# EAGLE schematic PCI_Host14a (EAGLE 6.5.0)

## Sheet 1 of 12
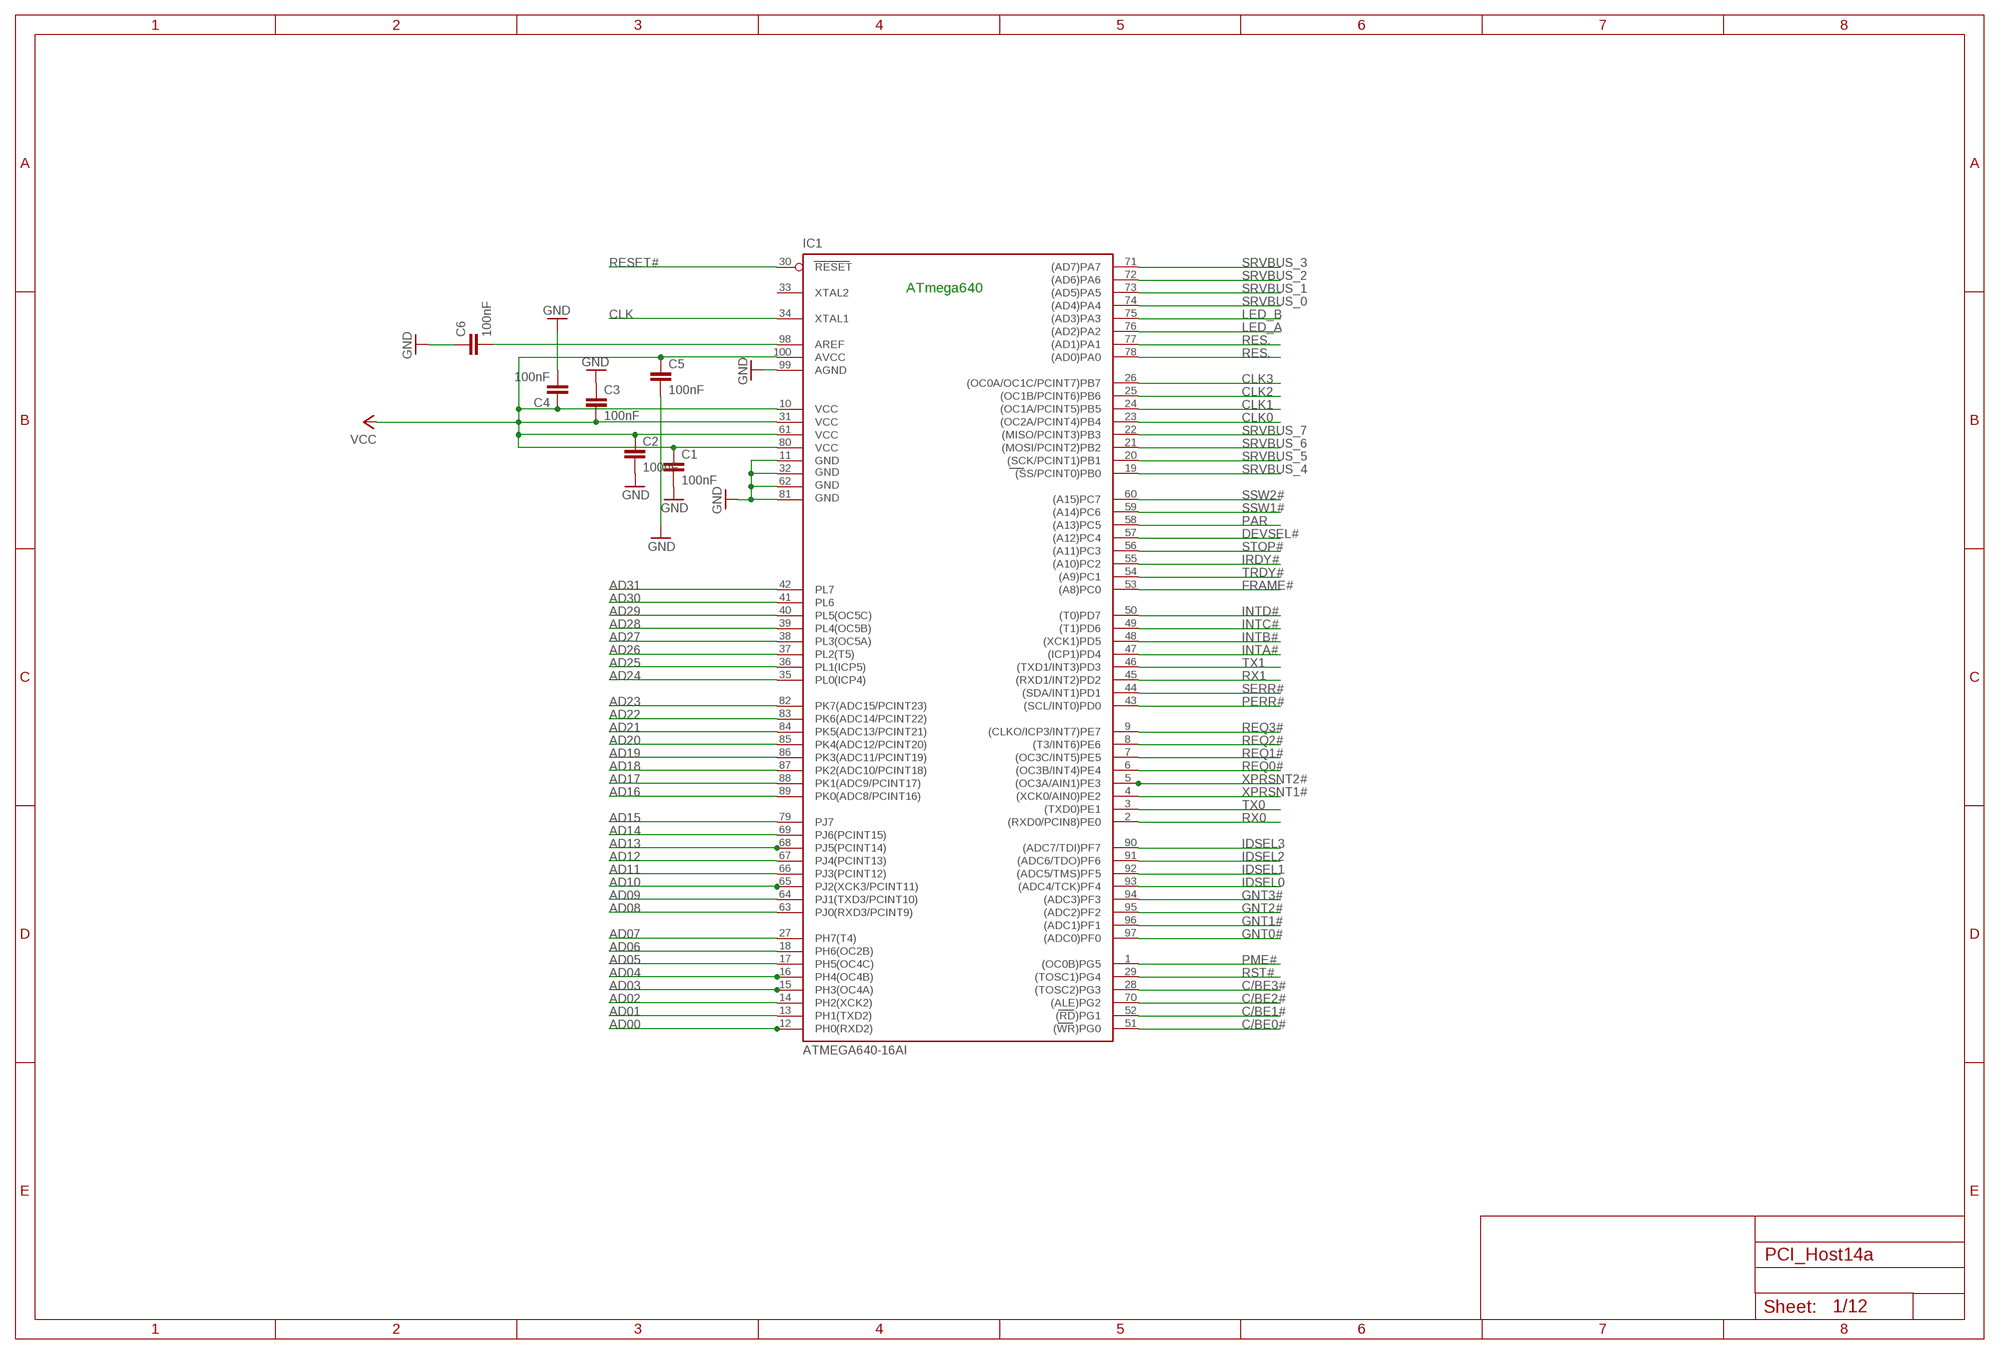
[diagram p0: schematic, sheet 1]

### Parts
C1  100nF  C-EU025-025X050  [C025-025X050]
C2  100nF  C-EU025-025X050  [C025-025X050]
C3  100nF  C-EU025-025X050  [C025-025X050]
C4  100nF  C-EU025-025X050  [C025-025X050]
C5  100nF  C-EU025-025X050  [C025-025X050]
C6  100nF  C-EU025-025X050  [C025-025X050]
IC1  ATMEGA640-16AI  [TQFP100]

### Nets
AD00: IC1.12(PH0(RXD2)) ; also sheet 8
AD01: IC1.13(PH1(TXD2)) ; also sheet 8
AD02: IC1.14(PH2(XCK2)) ; also sheet 8
AD03: IC1.15(PH3(OC4A)) ; also sheet 8
AD04: IC1.16(PH4(OC4B)) ; also sheet 8
AD05: IC1.17(PH5(OC4C)) ; also sheet 8
AD06: IC1.18(PH6(OC2B)) ; also sheet 8
AD07: IC1.27(PH7(T4)) ; also sheet 8
AD08: IC1.63(PJ0(RXD3/PCINT9)) ; also sheet 8
AD09: IC1.64(PJ1(TXD3/PCINT10)) ; also sheet 8
AD10: IC1.65(PJ2(XCK3/PCINT11)) ; also sheet 8
AD11: IC1.66(PJ3(PCINT12)) ; also sheet 8
AD12: IC1.67(PJ4(PCINT13)) ; also sheet 8
AD13: IC1.68(PJ5(PCINT14)) ; also sheet 8
AD14: IC1.69(PJ6(PCINT15)) ; also sheet 8
AD15: IC1.79(PJ7) ; also sheet 8
AD16: IC1.89(PK0(ADC8/PCINT16)) ; also sheet 8
AD17: IC1.88(PK1(ADC9/PCINT17)) ; also sheet 8
AD18: IC1.87(PK2(ADC10/PCINT18)) ; also sheet 8
AD19: IC1.86(PK3(ADC11/PCINT19)) ; also sheet 8
AD20: IC1.85(PK4(ADC12/PCINT20)) ; also sheet 8
AD21: IC1.84(PK5(ADC13/PCINT21)) ; also sheet 8
AD22: IC1.83(PK6(ADC14/PCINT22)) ; also sheet 8
AD23: IC1.82(PK7(ADC15/PCINT23)) ; also sheet 8
AD24: IC1.35(PL0(ICP4)) ; also sheet 8
AD25: IC1.36(PL1(ICP5)) ; also sheet 8
AD26: IC1.37(PL2(T5)) ; also sheet 8
AD27: IC1.38(PL3(OC5A)) ; also sheet 8
AD28: IC1.39(PL4(OC5B)) ; also sheet 8
AD29: IC1.40(PL5(OC5C)) ; also sheet 8
AD30: IC1.41(PL6) ; also sheet 8
AD31: IC1.42(PL7) ; also sheet 8
AREF: C6.2 IC1.98(AREF)
C/BE0#: IC1.51((WR)PG0) ; also sheet 8
C/BE1#: IC1.52((RD)PG1) ; also sheet 8
C/BE2#: IC1.70((ALE)PG2) ; also sheet 8
C/BE3#: IC1.28((TOSC2)PG3) ; also sheet 8
CLK: IC1.34(XTAL1) ; also sheet 3
CLK0: IC1.23((OC2A/PCINT4)PB4) ; also sheet 8
CLK1: IC1.24((OC1A/PCINT5)PB5) ; also sheet 8
CLK2: IC1.25((OC1B/PCINT6)PB6) ; also sheet 8
CLK3: IC1.26((OC0A/OC1C/PCINT7)PB7) ; also sheet 8
DEVSEL#: IC1.57((A12)PC4) ; also sheet 2,8
FRAME#: IC1.53((A8)PC0) ; also sheet 2,8
GND: C1.2 C2.2 C3.1 C4.2 C5.2 C6.1 IC1.11(GND) IC1.32(GND1) IC1.62(GND2) IC1.81(GND3) IC1.99(AGND) ; also sheet 2,3,4,5,6,7,8,12
GNT0#: IC1.97((ADC0)PF0) ; also sheet 8
GNT1#: IC1.96((ADC1)PF1) ; also sheet 8
GNT2#: IC1.95((ADC2)PF2) ; also sheet 8
GNT3#: IC1.94((ADC3)PF3) ; also sheet 8
IDSEL0: IC1.93((ADC4/TCK)PF4) ; also sheet 8
IDSEL1: IC1.92((ADC5/TMS)PF5) ; also sheet 8
IDSEL2: IC1.91((ADC6/TDO)PF6) ; also sheet 8
IDSEL3: IC1.90((ADC7/TDI)PF7) ; also sheet 8
INTA#: IC1.47((ICP1)PD4) ; also sheet 2,8
INTB#: IC1.48((XCK1)PD5) ; also sheet 2,8
INTC#: IC1.49((T1)PD6) ; also sheet 2,8
INTD#: IC1.50((T0)PD7) ; also sheet 2,8
IRDY#: IC1.55((A10)PC2) ; also sheet 2,8
LED_A: IC1.76((AD2)PA2) ; also sheet 6
LED_B: IC1.75((AD3)PA3) ; also sheet 6
PAR: IC1.58((A13)PC5) ; also sheet 8
PERR#: IC1.43((SCL/INT0)PD0) ; also sheet 2,8
PME#: IC1.1((OC0B)PG5) ; also sheet 8
REQ0#: IC1.6((OC3B/INT4)PE4) ; also sheet 8
REQ1#: IC1.7((OC3C/INT5)PE5) ; also sheet 8
REQ2#: IC1.8((T3/INT6)PE6) ; also sheet 8
REQ3#: IC1.9((CLKO/ICP3/INT7)PE7) ; also sheet 8
RES.: IC1.77((AD1)PA1) IC1.78((AD0)PA0)
RESET#: IC1.30(RESET) ; also sheet 3
RST#: IC1.29((TOSC1)PG4) ; also sheet 8
RX0: IC1.2((RXD0/PCIN8)PE0) ; also sheet 4
RX1: IC1.45((RXD1/INT2)PD2) ; also sheet 4,5
SERR#: IC1.44((SDA/INT1)PD1) ; also sheet 2,8
SRVBUS_0: IC1.74((AD4)PA4) ; also sheet 6
SRVBUS_1: IC1.73((AD5)PA5) ; also sheet 6
SRVBUS_2: IC1.72((AD6)PA6) ; also sheet 6
SRVBUS_3: IC1.71((AD7)PA7) ; also sheet 6
SRVBUS_4: IC1.19((SS/PCINT0)PB0) ; also sheet 6
SRVBUS_5: IC1.20((SCK/PCINT1)PB1) ; also sheet 3,6
SRVBUS_6: IC1.21((MOSI/PCINT2)PB2) ; also sheet 3,6
SRVBUS_7: IC1.22((MISO/PCINT3)PB3) ; also sheet 3,6
SSW1#: IC1.59((A14)PC6) ; also sheet 6
SSW2#: IC1.60((A15)PC7) ; also sheet 6
STOP#: IC1.56((A11)PC3) ; also sheet 2,8
TRDY#: IC1.54((A9)PC1) ; also sheet 2,8
TX0: IC1.3((TXD0)PE1) ; also sheet 4
TX1: IC1.46((TXD1/INT3)PD3) ; also sheet 4,5
VCC: C1.1 C2.1 C3.2 C4.1 C5.1 IC1.10(VCC) IC1.31(VCC1) IC1.61(VCC2) IC1.80(VCC3) IC1.100(AVCC) ; also sheet 2,3,4,5,6,7,12
XPRSNT1#: IC1.4((XCK0/AIN0)PE2) ; also sheet 2
XPRSNT2#: IC1.5((OC3A/AIN1)PE3) ; also sheet 2
Unconnected: IC1.33(XTAL2)

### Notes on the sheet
- ATmega640

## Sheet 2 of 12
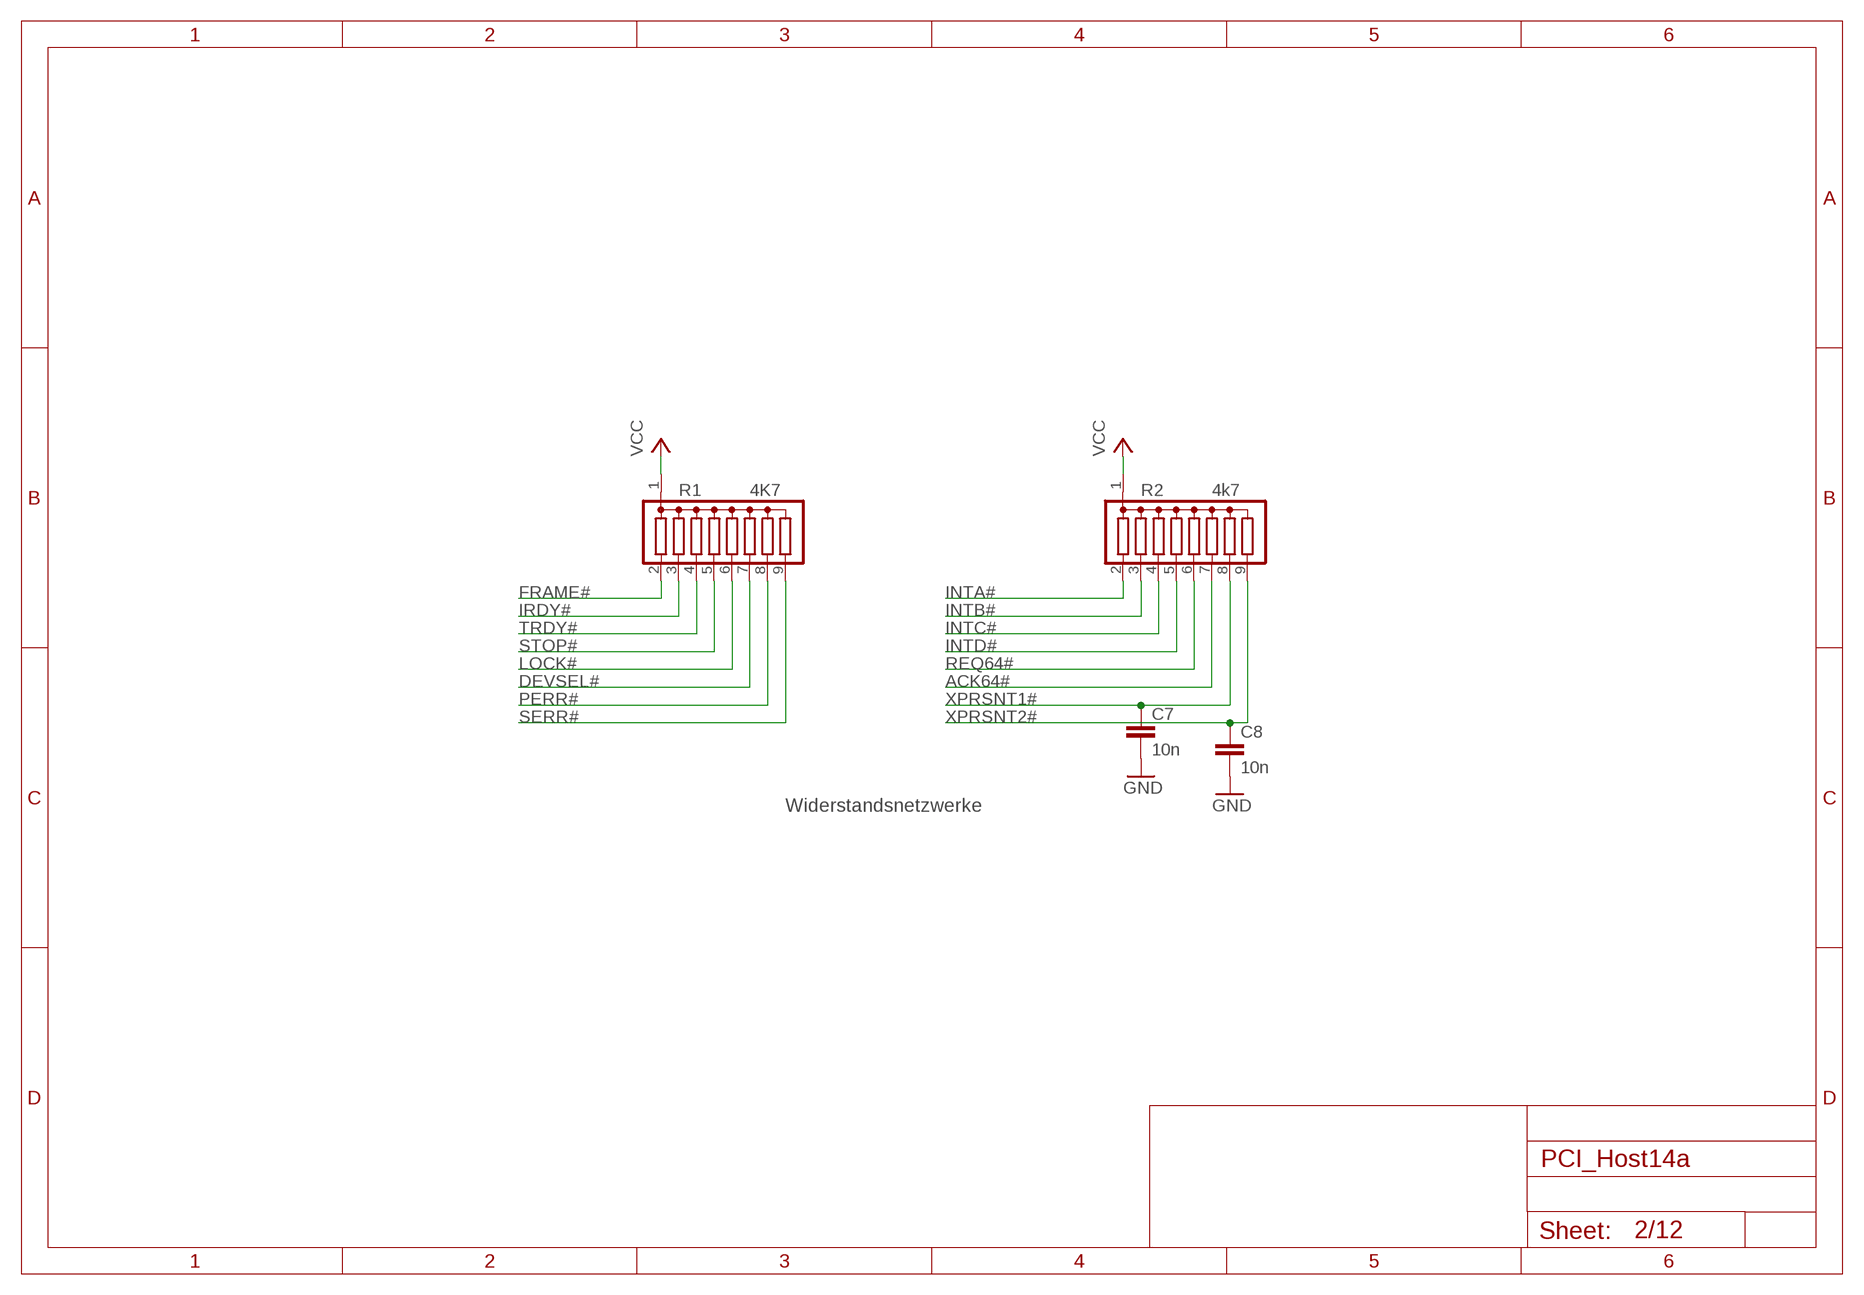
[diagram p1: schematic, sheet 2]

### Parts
C7  10n  C-EU025-025X050  [C025-025X050]
C8  10n  C-EU025-025X050  [C025-025X050]
R1  4K7  G08R  [SIL9]
R2  4k7  G08R  [SIL9]

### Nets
ACK64#: R2.7
DEVSEL#: R1.7 ; also sheet 1,8
FRAME#: R1.2 ; also sheet 1,8
GND: C7.2 C8.2 ; also sheet 1,3,4,5,6,7,8,12
INTA#: R2.2 ; also sheet 1,8
INTB#: R2.3 ; also sheet 1,8
INTC#: R2.4 ; also sheet 1,8
INTD#: R2.5 ; also sheet 1,8
IRDY#: R1.3 ; also sheet 1,8
LOCK#: R1.6 ; also sheet 8
PERR#: R1.8 ; also sheet 1,8
REQ64#: R2.6
SERR#: R1.9 ; also sheet 1,8
STOP#: R1.5 ; also sheet 1,8
TRDY#: R1.4 ; also sheet 1,8
VCC: R1.1 R2.1 ; also sheet 1,3,4,5,6,7,12
XPRSNT1#: C7.1 R2.8 ; also sheet 1
XPRSNT2#: C8.1 R2.9 ; also sheet 1

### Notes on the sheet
- Widerstandsnetzwerke

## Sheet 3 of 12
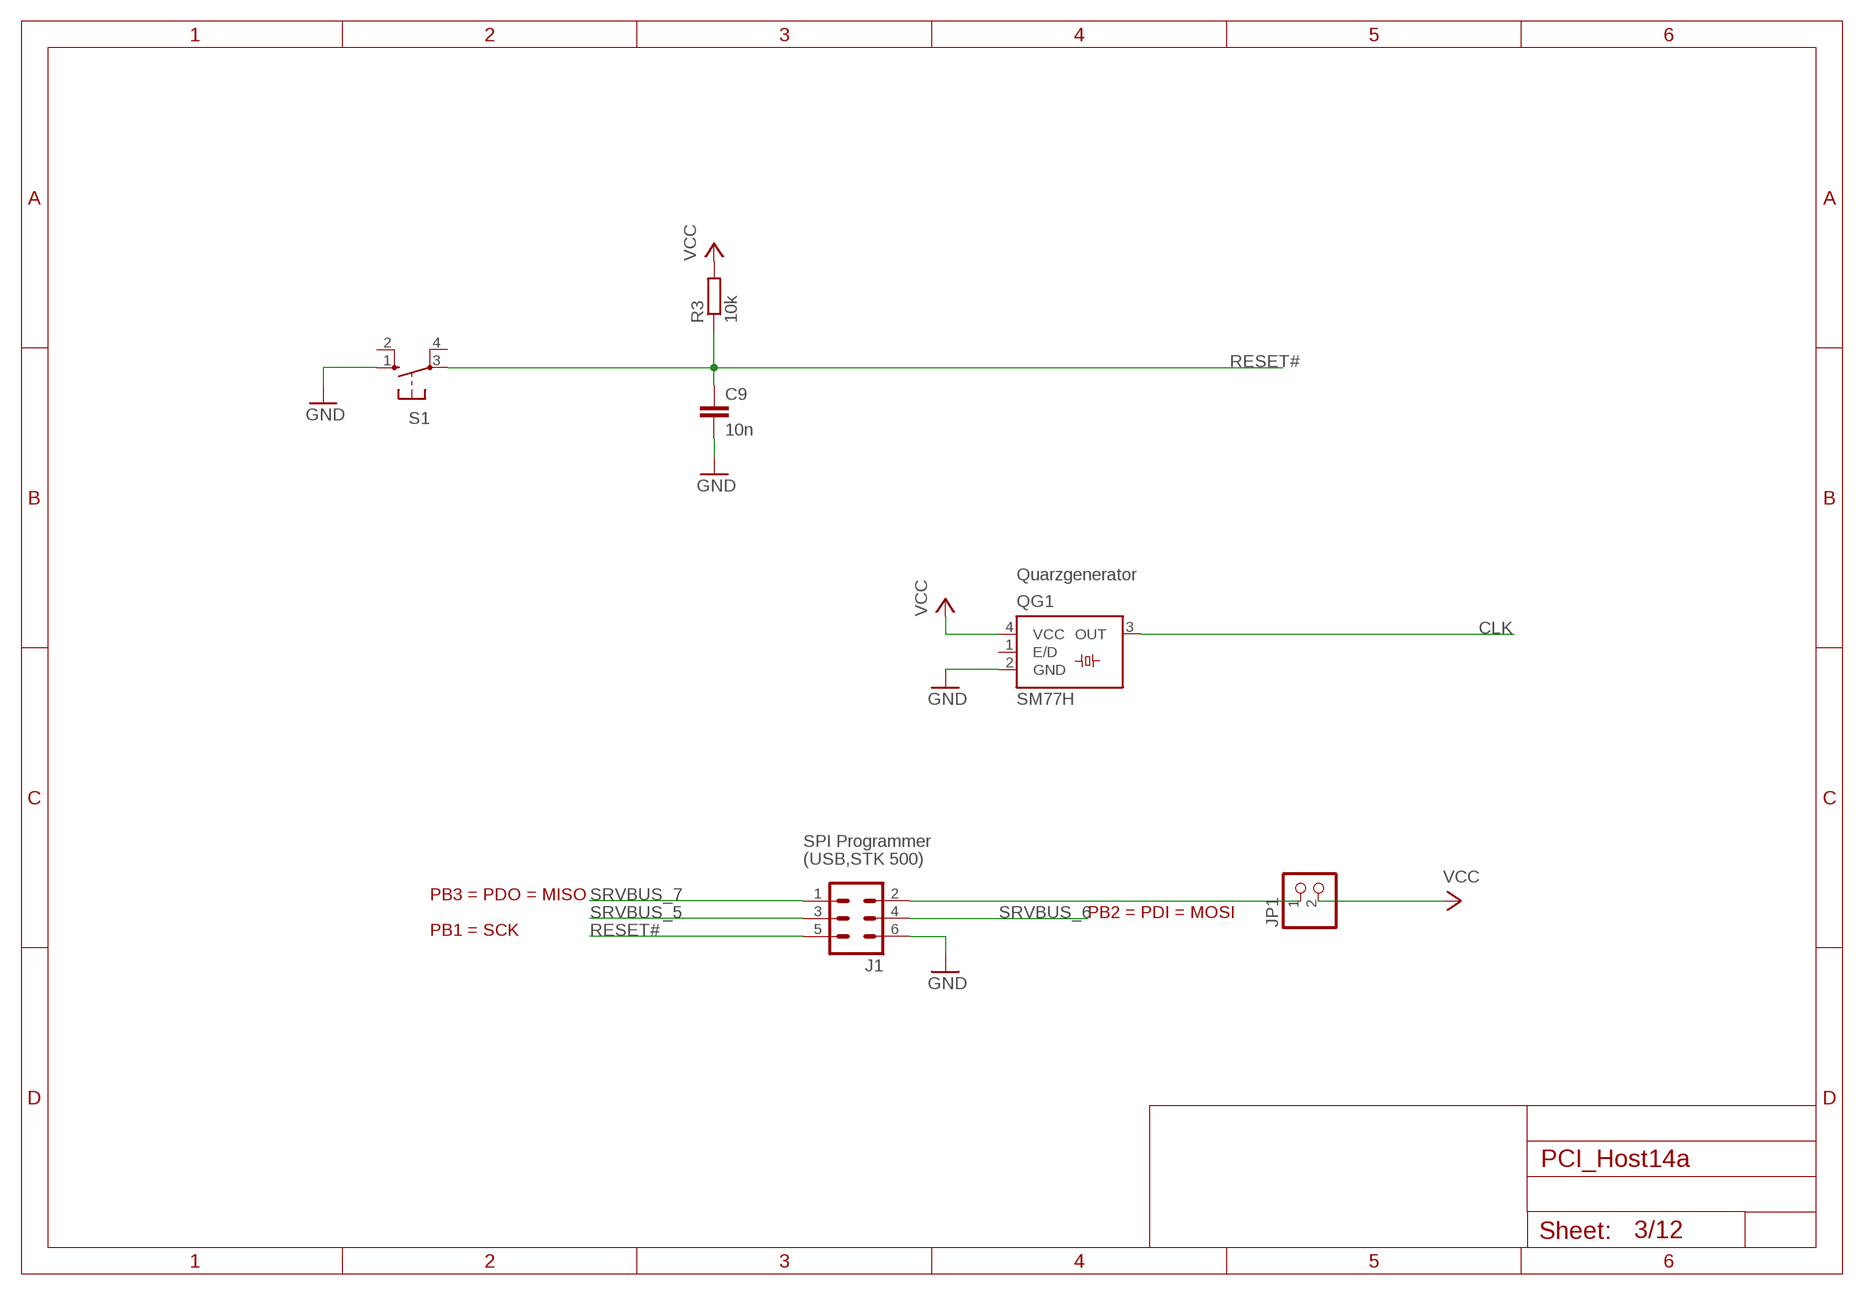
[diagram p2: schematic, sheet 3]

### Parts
C9  10n  C-EU025-025X050  [C025-025X050]
J1  ML6  [ML6]
JP1  PINHD-1X2  [1X02]
QG1  SM77H  [SM77H]
R3  10k  R-EU_0207/10  [0207/10]
S1  10-XX  [B3F-10XX]

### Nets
CLK: QG1.3(OUT) ; also sheet 1
GND: C9.2 J1.6 QG1.2(GND) S1.1(S) ; also sheet 1,2,4,5,6,7,8,12
N$14: J1.2 JP1.1
RESET#: C9.1 J1.5 R3.1 S1.3(P) ; also sheet 1
SRVBUS_5: J1.3 ; also sheet 1,6
SRVBUS_6: J1.4 ; also sheet 1,6
SRVBUS_7: J1.1 ; also sheet 1,6
VCC: JP1.2 QG1.4(VCC) R3.2 ; also sheet 1,2,4,5,6,7,12
Unconnected: QG1.1(E/D) S1.2(S1) S1.4(P1)

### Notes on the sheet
- Quarzgenerator
- SPI Programmer
- (USB,STK 500)
- PB3 = PDO = MISO
- PB2 = PDI = MOSI
- PB1 = SCK

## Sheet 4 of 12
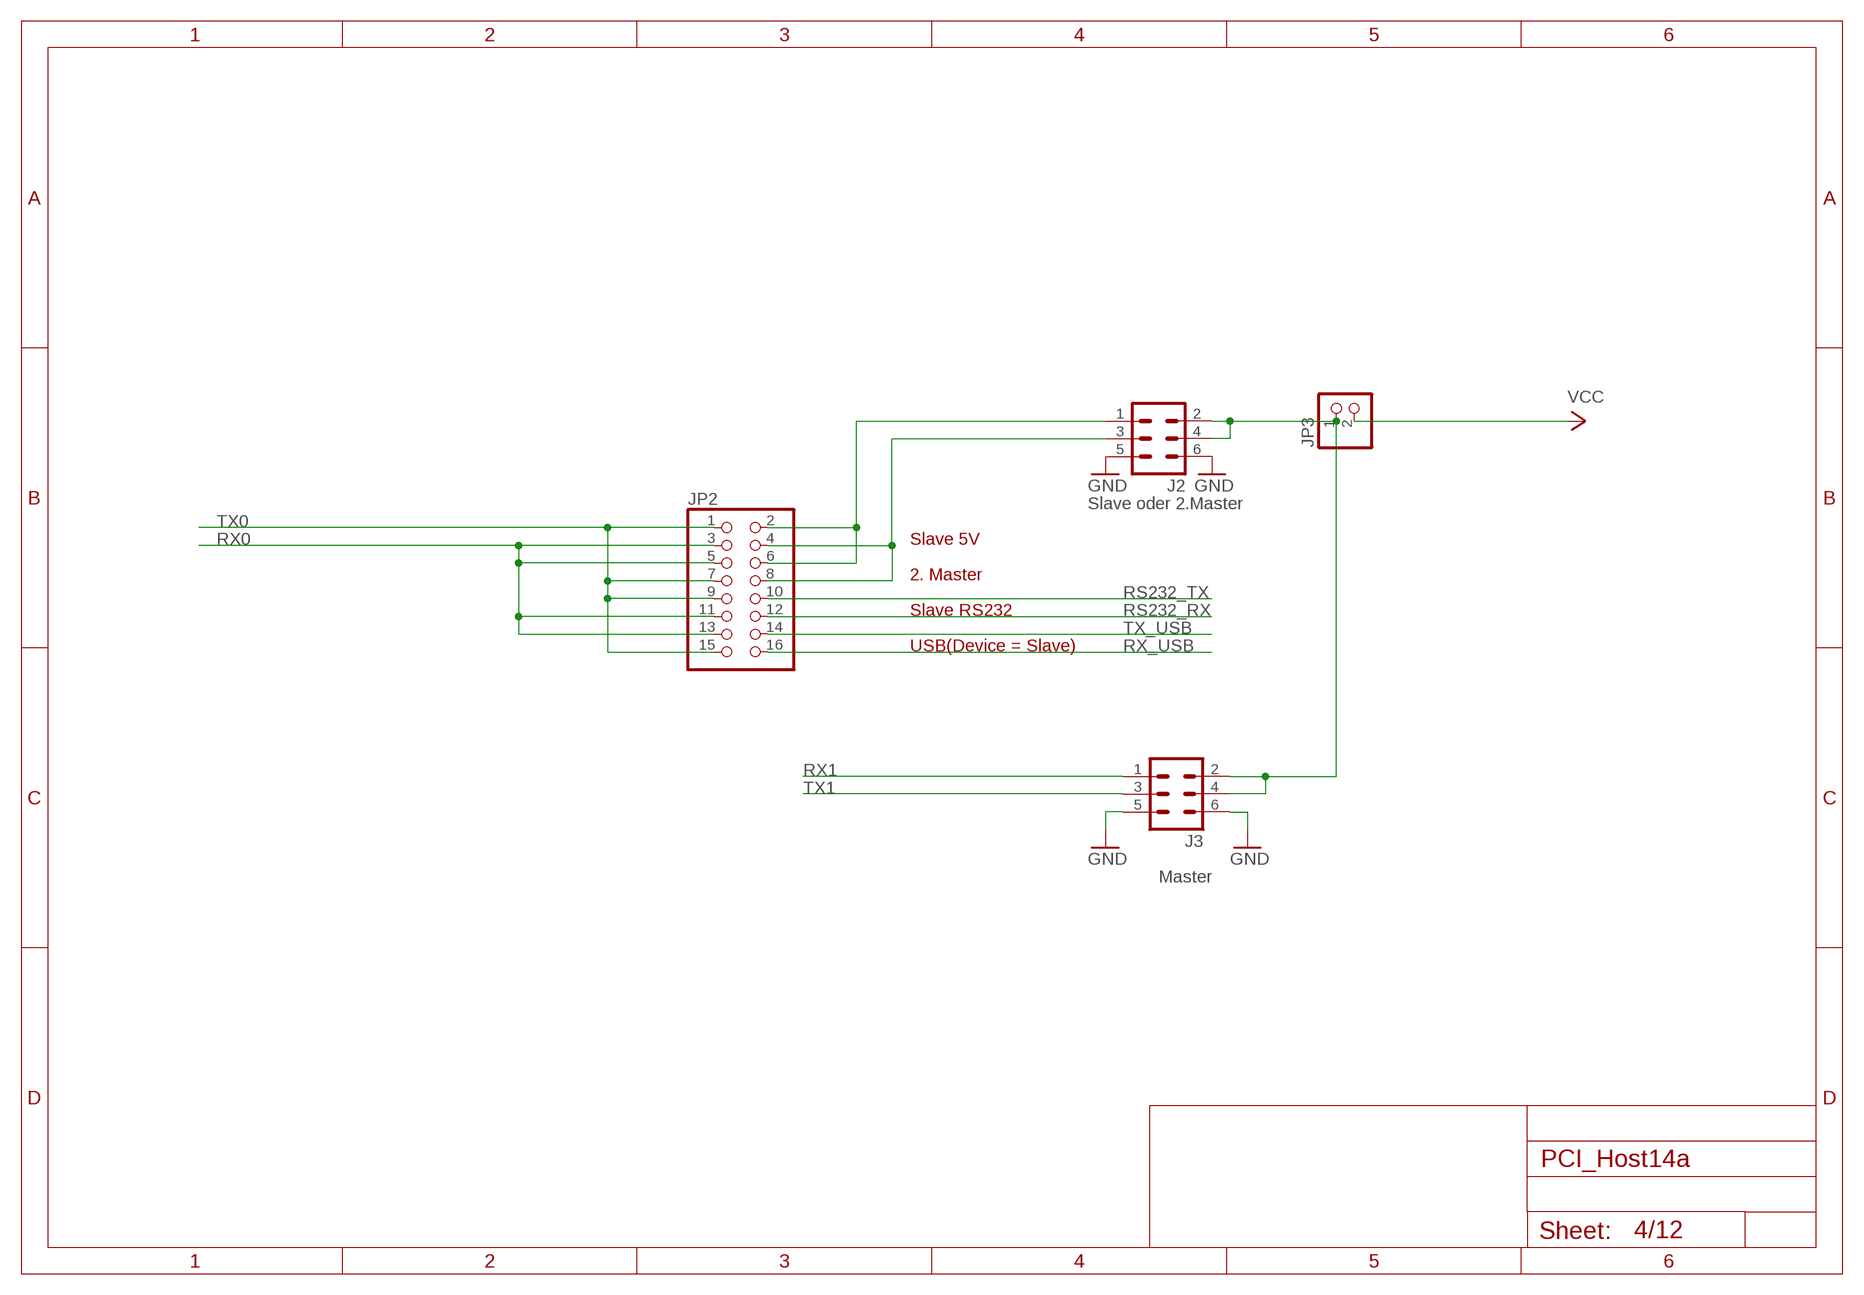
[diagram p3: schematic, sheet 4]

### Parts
J2  ML6  [ML6]
J3  ML6  [ML6]
JP2  PINHD-2X8  [2X08]
JP3  PINHD-1X2  [1X02]

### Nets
GND: J2.5 J2.6 J3.5 J3.6 ; also sheet 1,2,3,5,6,7,8,12
N$3: J2.2 J2.4 J3.2 J3.4 JP3.1
N$15: J2.3 JP2.4 JP2.8
N$101: J2.1 JP2.2 JP2.6
RS232_RX: JP2.12 ; also sheet 5
RS232_TX: JP2.10 ; also sheet 5
RX0: JP2.3 JP2.5 JP2.11 JP2.13 ; also sheet 1
RX1: J3.1 ; also sheet 1,5
RX_USB: JP2.16 ; also sheet 7
TX0: JP2.1 JP2.7 JP2.9 JP2.15 ; also sheet 1
TX1: J3.3 ; also sheet 1,5
TX_USB: JP2.14 ; also sheet 7
VCC: JP3.2 ; also sheet 1,2,3,5,6,7,12

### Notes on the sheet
- Slave oder 2.Master
- Slave 5V
- 2. Master
- Slave RS232
- USB(Device = Slave)
- Master

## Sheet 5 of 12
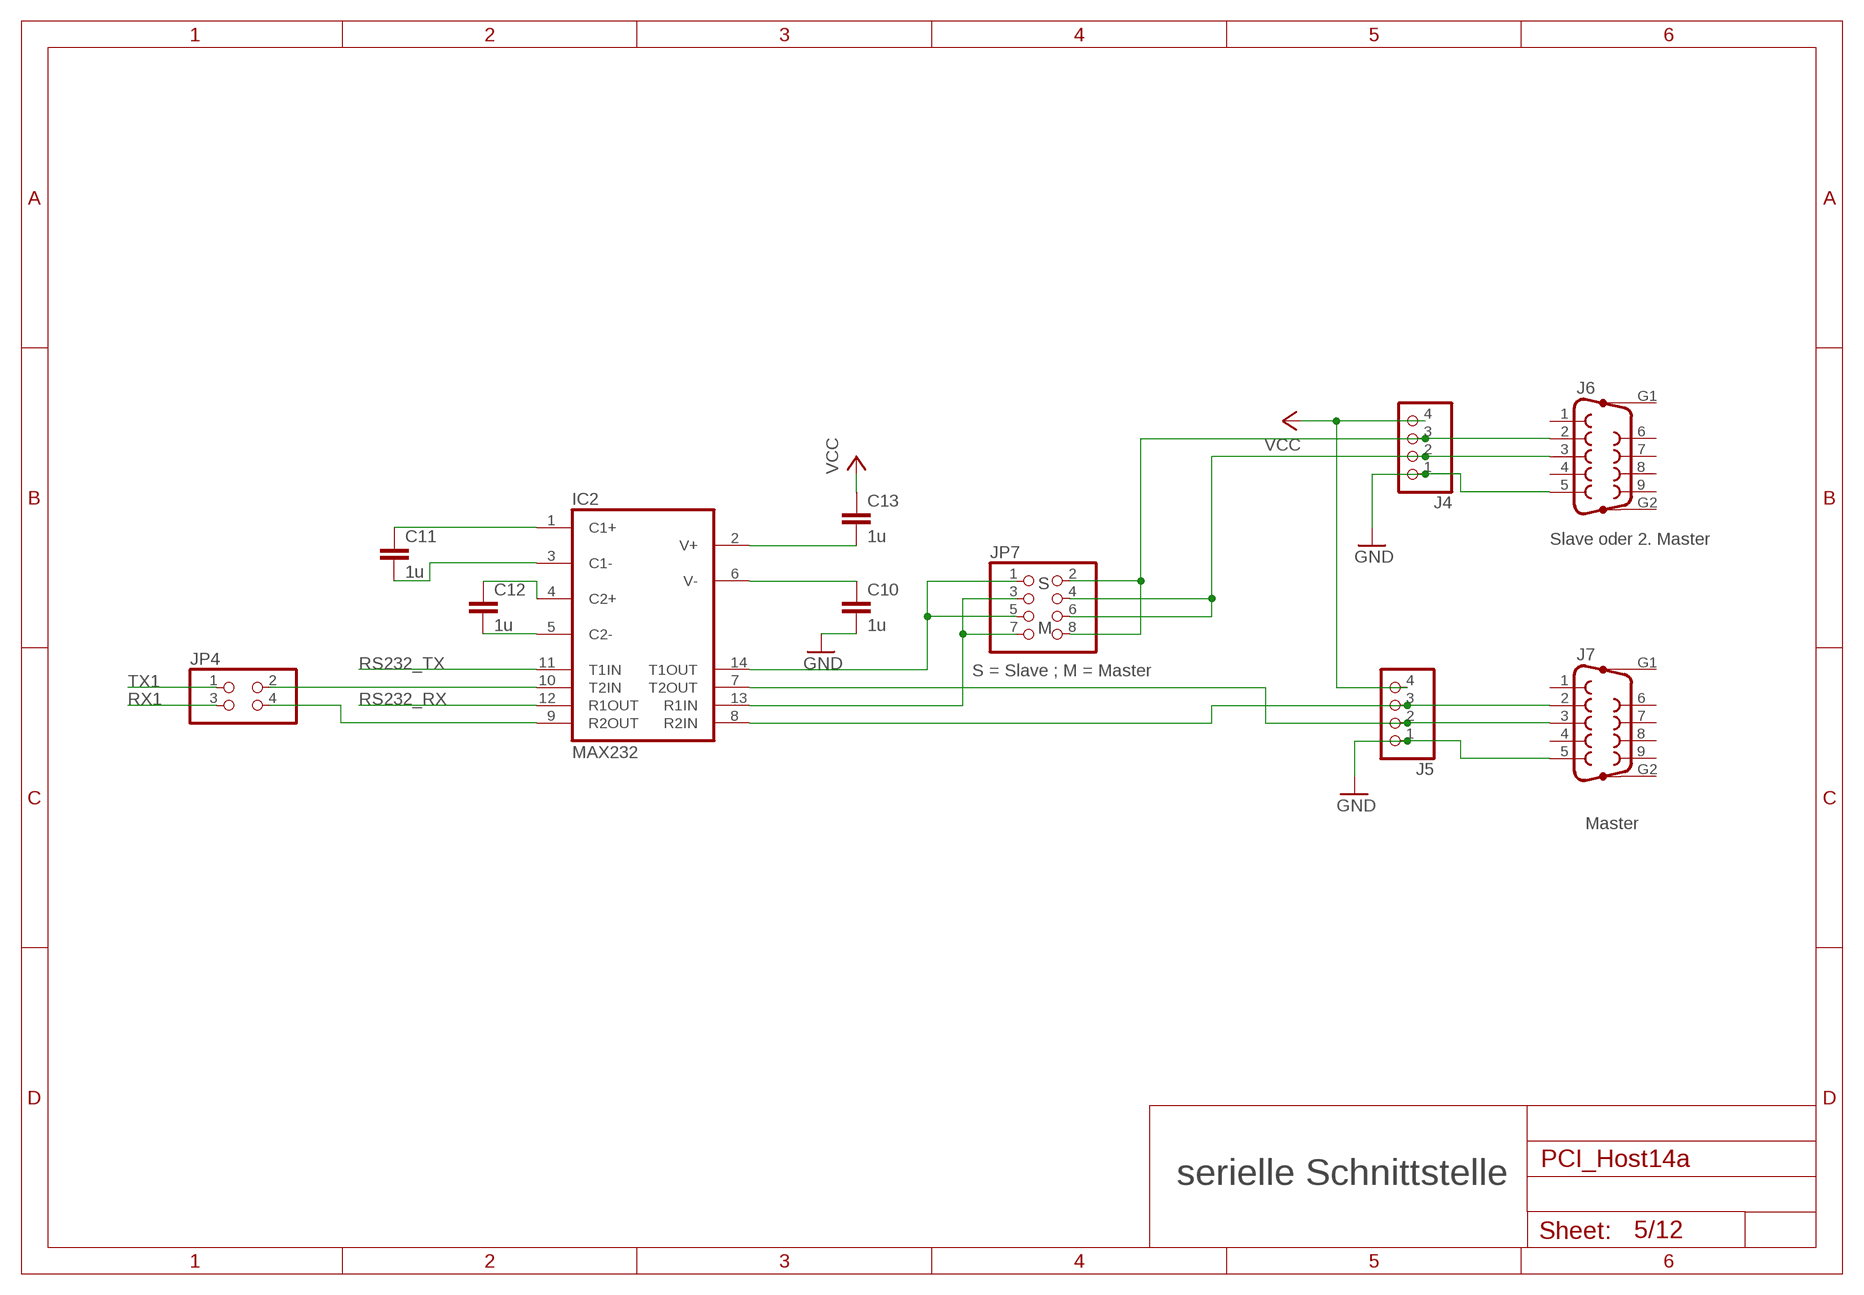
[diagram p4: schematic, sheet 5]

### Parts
C10  1u  C-EU025-025X050  [C025-025X050]
C11  1u  C-EU025-025X050  [C025-025X050]
C12  1u  C-EU025-025X050  [C025-025X050]
C13  1u  C-EU025-025X050  [C025-025X050]
IC2  MAX232  [DIL16]
J4  PINHD-1X4  [1X04]
J5  PINHD-1X4  [1X04]
J6  F09HP  [F09HP]
J7  F09HP  [F09HP]
JP4  PINHD-2X2  [2X02]
JP7  PINHD-2X4  [2X04]

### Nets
GND: C10.2 J4.1 J5.1 J6.5 J7.5 ; also sheet 1,2,3,4,6,7,8,12
N$9: C11.1 IC2.1(C1+)
N$11: C11.2 IC2.3(C1-)
N$13: C12.1 IC2.4(C2+)
N$16: C12.2 IC2.5(C2-)
N$17: C13.2 IC2.2(V+)
N$18: IC2.10(T2IN) JP4.2
N$19: IC2.9(R2OUT) JP4.4
N$21: C10.1 IC2.6(V-)
N$22: IC2.14(T1OUT) JP7.1 JP7.5
N$23: IC2.13(R1IN) JP7.3 JP7.7
N$24: J4.3 J6.2 JP7.2 JP7.8
N$26: J4.2 J6.3 JP7.4 JP7.6
N$27: IC2.7(T2OUT) J5.2 J7.3
N$28: IC2.8(R2IN) J5.3 J7.2
RS232_RX: IC2.12(R1OUT) ; also sheet 4
RS232_TX: IC2.11(T1IN) ; also sheet 4
RX1: JP4.3 ; also sheet 1,4
TX1: JP4.1 ; also sheet 1,4
VCC: C13.1 J4.4 J5.4 ; also sheet 1,2,3,4,6,7,12
Unconnected: J6.1 J6.4 J6.6 J6.7 J6.8 J6.9 J6.G1 J6.G2 J7.1 J7.4 J7.6 J7.7 J7.8 J7.9 J7.G1 J7.G2

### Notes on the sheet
- Slave oder 2. Master
- S
- M
- S = Slave ; M = Master
- Master
- serielle Schnittstelle

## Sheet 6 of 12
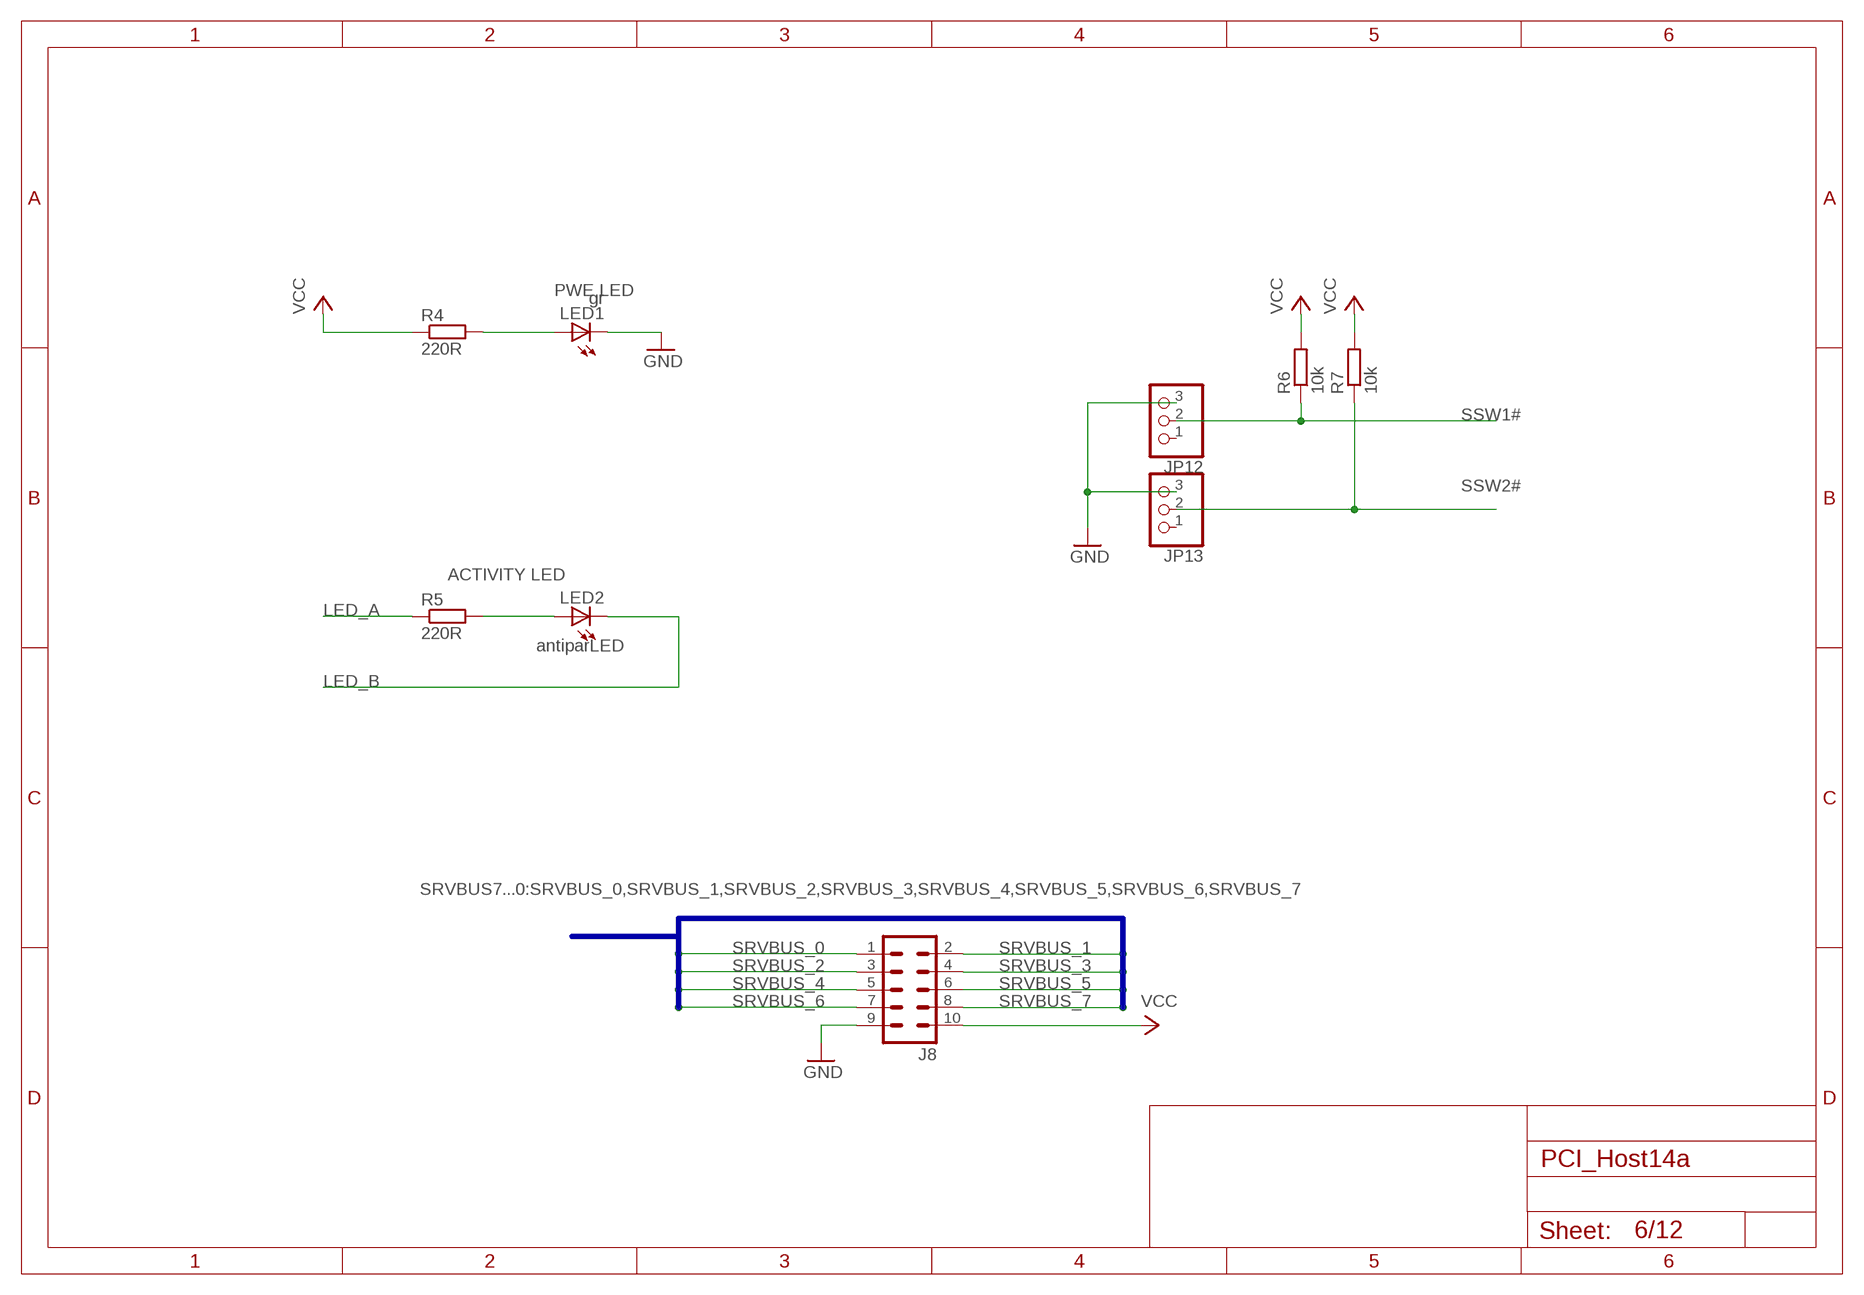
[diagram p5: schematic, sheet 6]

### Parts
J8  ML10  [ML10]
JP12  PINHD-1X3  [1X03]
JP13  PINHD-1X3  [1X03]
LED1  gr  LEDSMT1206  [1206]
LED2  LEDSMT1206  [1206]
R4  220R  R-EU_0207/10  [0207/10]
R5  220R  R-EU_0207/10  [0207/10]
R6  10k  R-EU_0207/10  [0207/10]
R7  10k  R-EU_0207/10  [0207/10]

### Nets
GND: J8.9 JP12.3 JP13.3 LED1.C ; also sheet 1,2,3,4,5,7,8,12
LED_A: R5.1 ; also sheet 1
LED_B: LED2.C ; also sheet 1
N$2: LED2.A R5.2
N$33: LED1.A R4.2
SRVBUS_0: J8.1 ; also sheet 1
SRVBUS_1: J8.2 ; also sheet 1
SRVBUS_2: J8.3 ; also sheet 1
SRVBUS_3: J8.4 ; also sheet 1
SRVBUS_4: J8.5 ; also sheet 1
SRVBUS_5: J8.6 ; also sheet 1,3
SRVBUS_6: J8.7 ; also sheet 1,3
SRVBUS_7: J8.8 ; also sheet 1,3
SSW1#: JP12.2 R6.1 ; also sheet 1
SSW2#: JP13.2 R7.1 ; also sheet 1
VCC: J8.10 R4.1 R6.2 R7.2 ; also sheet 1,2,3,4,5,7,12
Unconnected: JP12.1 JP13.1

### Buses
SRVBUS7...0:SRVBUS_0,SRVBUS_1,SRVBUS_2,SRVBUS_3,SRVBUS_4,SRVBUS_5,SRVBUS_6,SRVBUS_7

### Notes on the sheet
- PWE LED
- ACTIVITY LED
- antiparLED

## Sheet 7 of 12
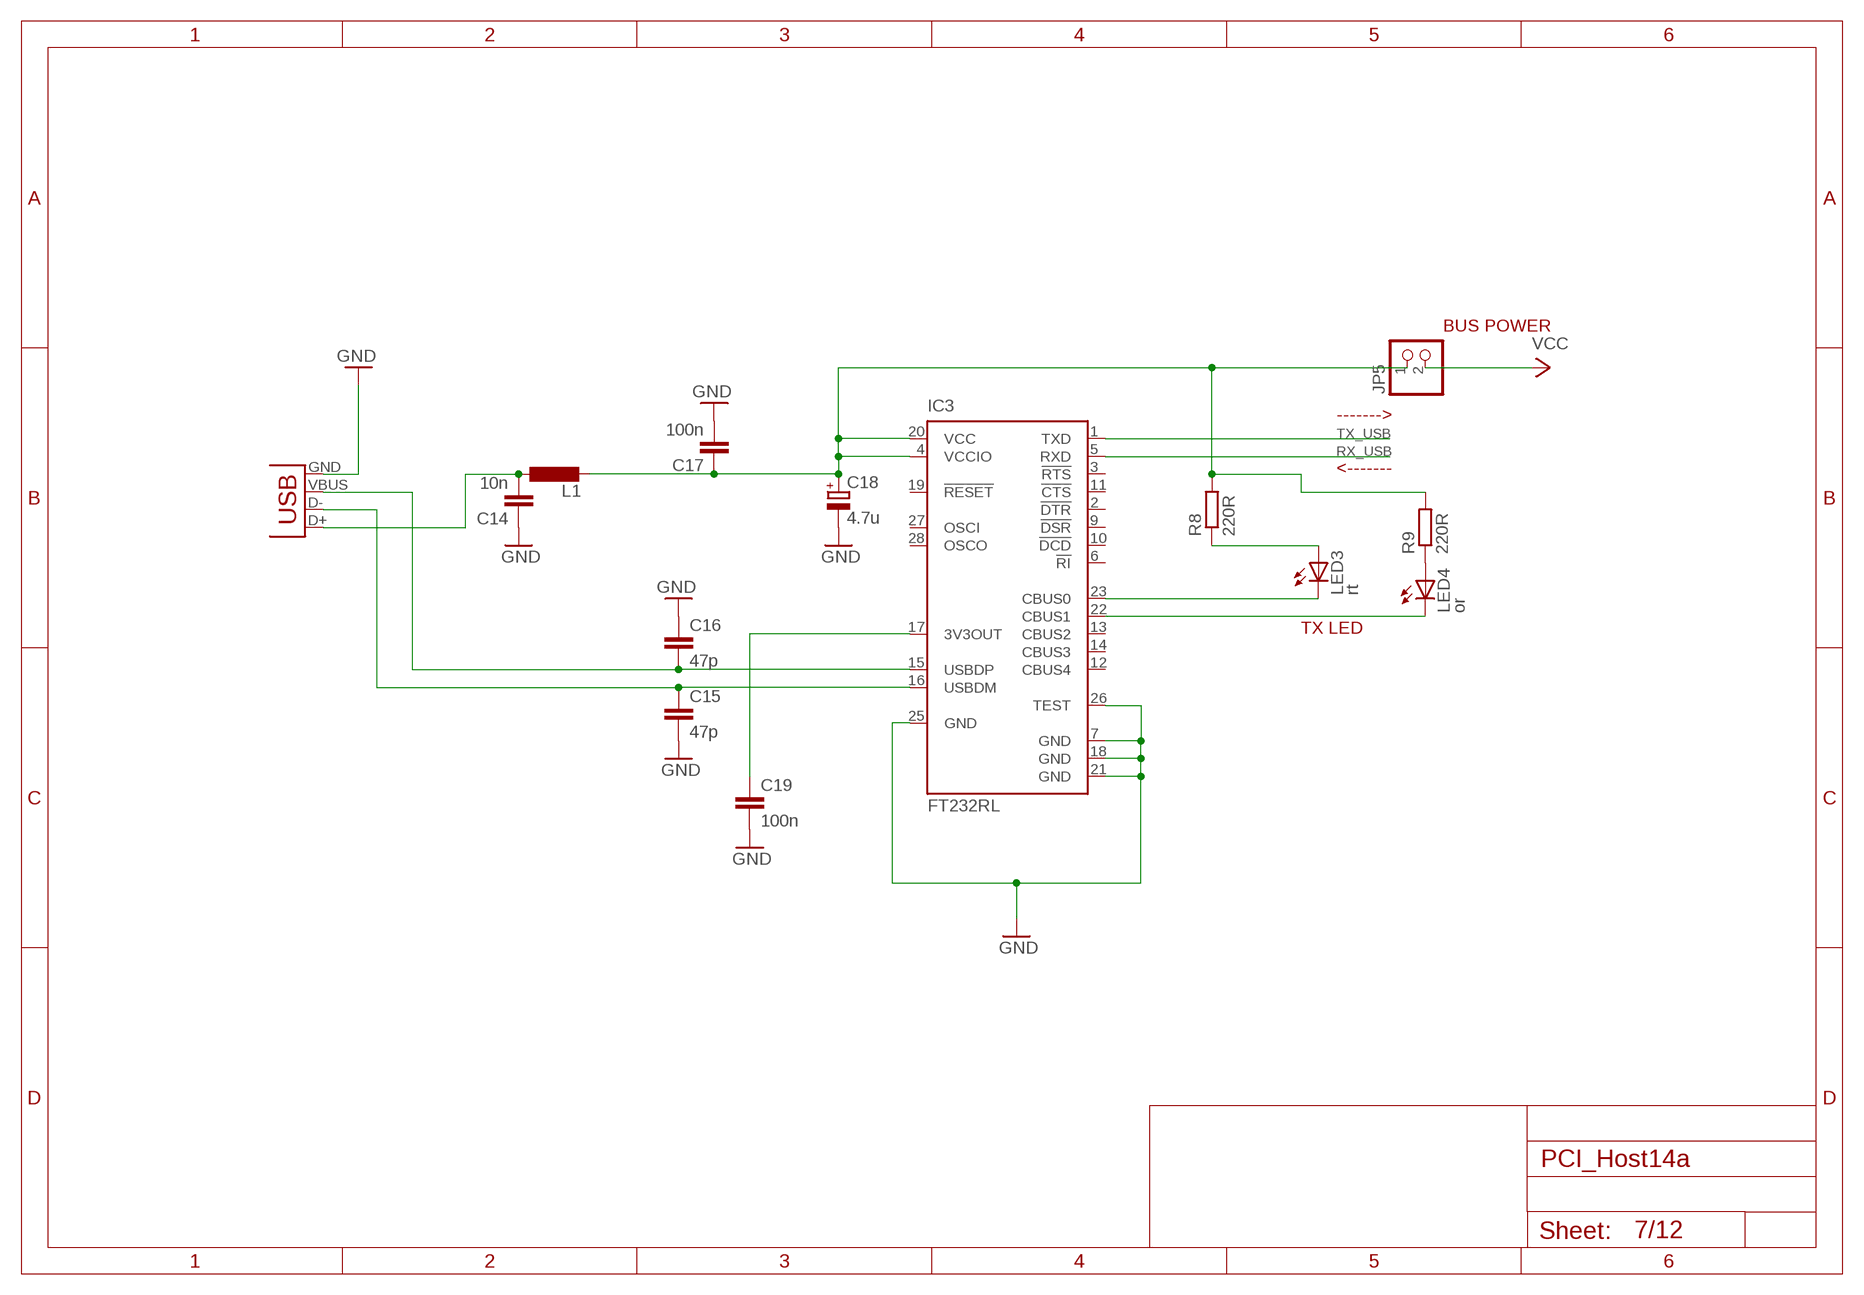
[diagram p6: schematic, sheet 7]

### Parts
C14  10n  C-EU025-025X050  [C025-025X050]
C15  47p  C-EU025-025X050  [C025-025X050]
C16  47p  C-EU025-025X050  [C025-025X050]
C17  100n  C-EU025-025X050  [C025-025X050]
C18  4.7u  CPOL-EUE2.5-6  [E2,5-6]
C19  100n  C-EU025-025X050  [C025-025X050]
IC3  FT232RL  [SSOP28]
JP5  PINHD-1X2  [1X02]
L1  L-EU  [M0805]
LED3  rt  LEDSMT1206  [1206]
LED4  or  LEDSMT1206  [1206]
R8  220R  R-EU_0207/10  [0207/10]
R9  220R  R-EU_0207/10  [0207/10]
X2  USB-MB-S  [USB-MB-S]

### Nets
GND: C14.1 C15.2 C16.1 C17.2 C18.- C19.2 IC3.7(GND) IC3.18(GND) IC3.21(GND) IC3.25(GND) IC3.26(TEST) X2.GND ; also sheet 1,2,3,4,5,6,8,12
N$4: C17.1 C18.+ IC3.4(VCCIO) IC3.20(VCC) JP5.1 L1.2 R8.2 R9.2
N$5: LED3.A R8.1
N$35: C15.1 IC3.16(USBDM) X2.D-
N$37: C19.1 IC3.17(3V3OUT)
N$38: IC3.22(CBUS1) LED4.C
N$39: IC3.23(CBUS0) LED3.C
N$40: C14.2 L1.1 X2.D+
N$41: LED4.A R9.1
N$46: C16.2 IC3.15(USBDP) X2.VBUS
RX_USB: IC3.5(RXD) ; also sheet 4
TX_USB: IC3.1(TXD) ; also sheet 4
VCC: JP5.2 ; also sheet 1,2,3,4,5,6,12
Unconnected: IC3.2(!DTR) IC3.3(!RTS) IC3.6(!RI) IC3.9(!DSR) IC3.10(!DCD) IC3.11(!CTS) IC3.12(CBUS4) IC3.13(CBUS2) IC3.14(CBUS3) IC3.19(!RESET) IC3.27(OSCI) IC3.28(OSCO)

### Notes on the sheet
- BUS POWER
- ------->
- <-------
- TX LED

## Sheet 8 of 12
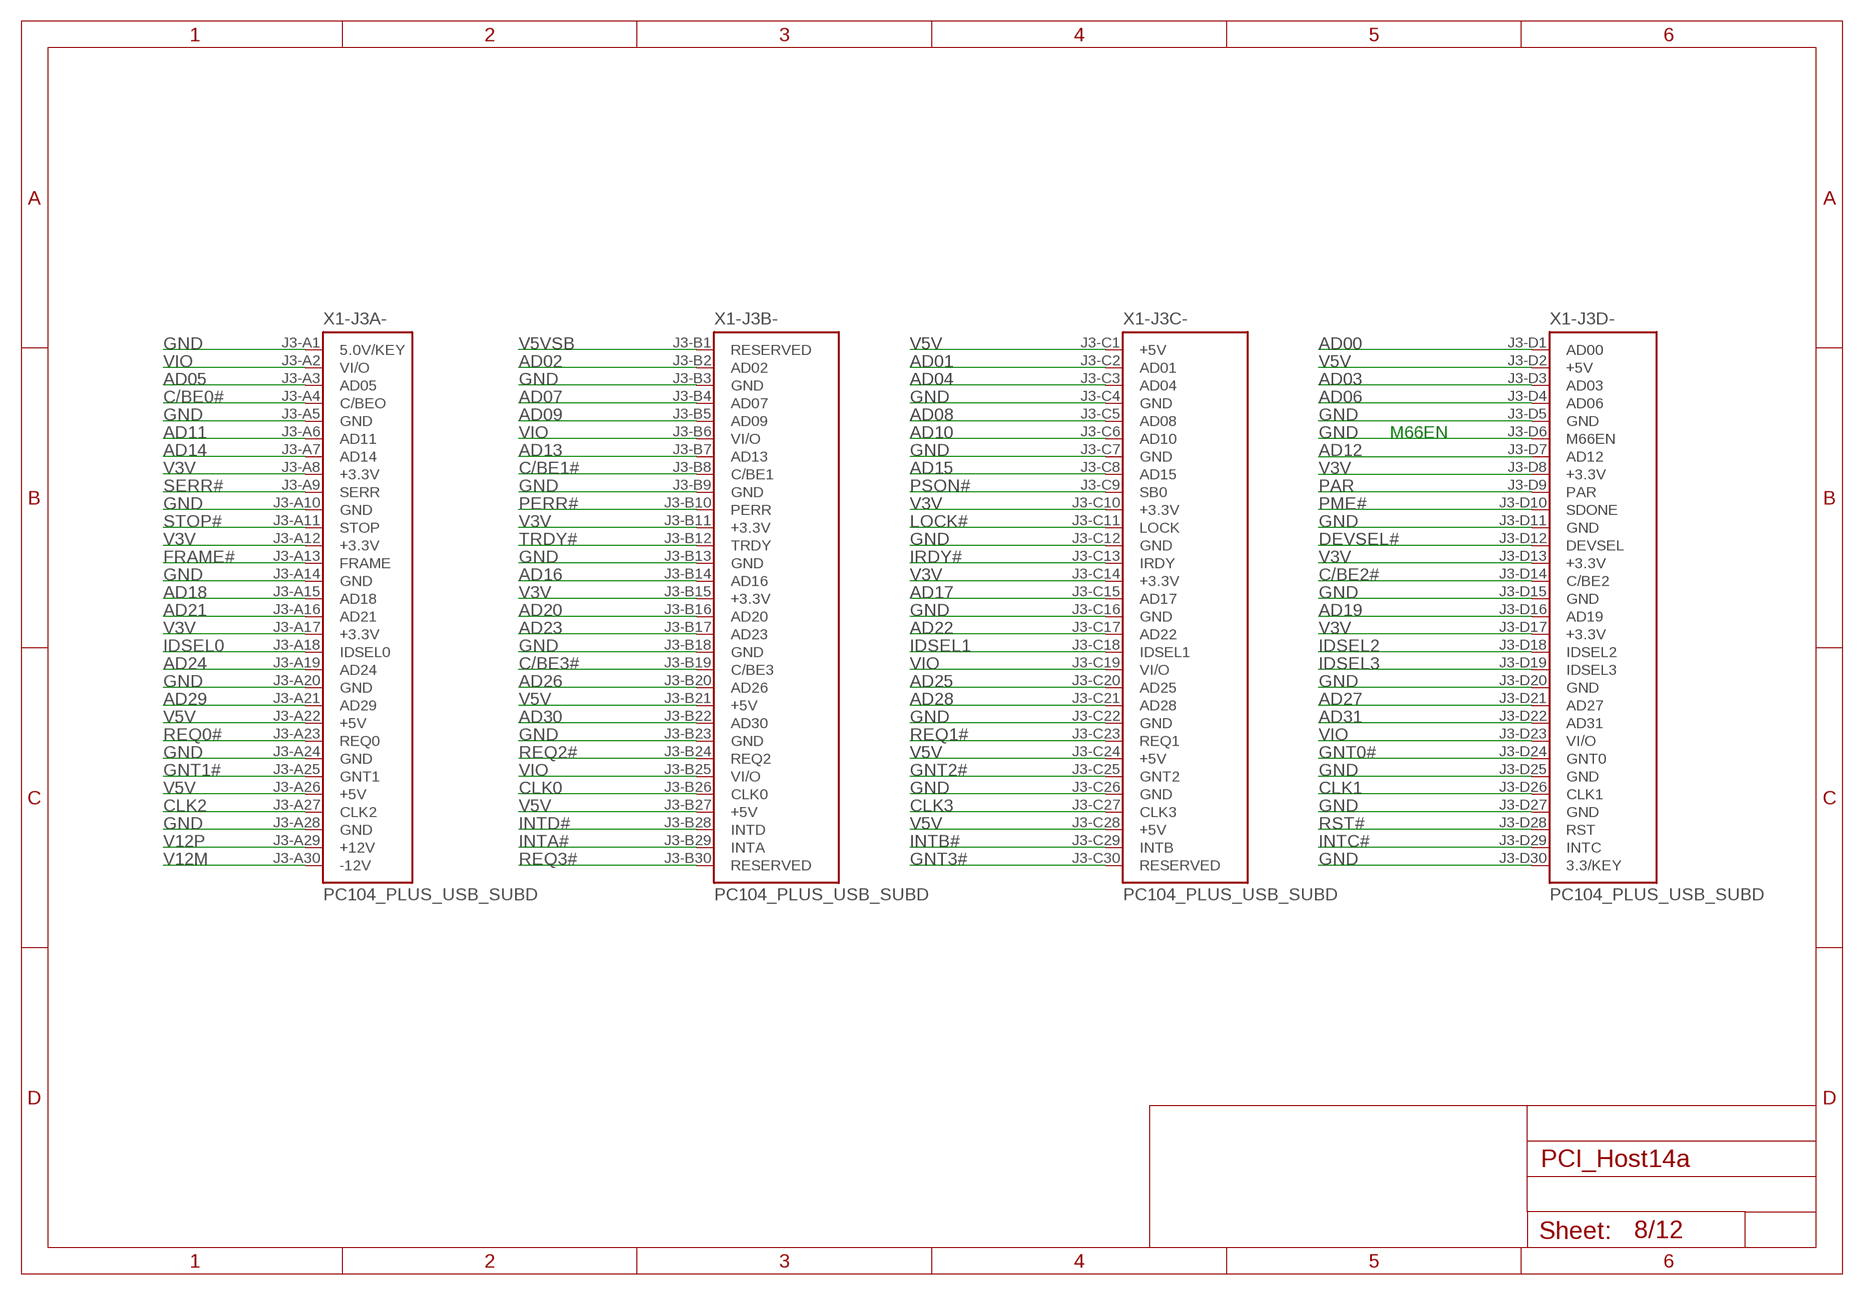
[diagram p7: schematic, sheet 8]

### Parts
X1  PC104_PLUS_USB_SUBD  [PC104-PLUS]

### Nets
AD00: X1.J3-D1(-J3D-:AD00) ; also sheet 1
AD01: X1.J3-C2(-J3C-:AD01) ; also sheet 1
AD02: X1.J3-B2(-J3B-:AD02) ; also sheet 1
AD03: X1.J3-D3(-J3D-:AD03) ; also sheet 1
AD04: X1.J3-C3(-J3C-:AD04) ; also sheet 1
AD05: X1.J3-A3(-J3A-:AD05) ; also sheet 1
AD06: X1.J3-D4(-J3D-:AD06) ; also sheet 1
AD07: X1.J3-B4(-J3B-:AD07) ; also sheet 1
AD08: X1.J3-C5(-J3C-:AD08) ; also sheet 1
AD09: X1.J3-B5(-J3B-:AD09) ; also sheet 1
AD10: X1.J3-C6(-J3C-:AD10) ; also sheet 1
AD11: X1.J3-A6(-J3A-:AD11) ; also sheet 1
AD12: X1.J3-D7(-J3D-:AD12) ; also sheet 1
AD13: X1.J3-B7(-J3B-:AD13) ; also sheet 1
AD14: X1.J3-A7(-J3A-:AD14) ; also sheet 1
AD15: X1.J3-C8(-J3C-:AD15) ; also sheet 1
AD16: X1.J3-B14(-J3B-:AD16) ; also sheet 1
AD17: X1.J3-C15(-J3C-:AD17) ; also sheet 1
AD18: X1.J3-A15(-J3A-:AD18) ; also sheet 1
AD19: X1.J3-D16(-J3D-:AD19) ; also sheet 1
AD20: X1.J3-B16(-J3B-:AD20) ; also sheet 1
AD21: X1.J3-A16(-J3A-:AD21) ; also sheet 1
AD22: X1.J3-C17(-J3C-:AD22) ; also sheet 1
AD23: X1.J3-B17(-J3B-:AD23) ; also sheet 1
AD24: X1.J3-A19(-J3A-:AD24) ; also sheet 1
AD25: X1.J3-C20(-J3C-:AD25) ; also sheet 1
AD26: X1.J3-B20(-J3B-:AD26) ; also sheet 1
AD27: X1.J3-D21(-J3D-:AD27) ; also sheet 1
AD28: X1.J3-C21(-J3C-:AD28) ; also sheet 1
AD29: X1.J3-A21(-J3A-:AD29) ; also sheet 1
AD30: X1.J3-B22(-J3B-:AD30) ; also sheet 1
AD31: X1.J3-D22(-J3D-:AD31) ; also sheet 1
C/BE0#: X1.J3-A4(-J3A-:C/BEO) ; also sheet 1
C/BE1#: X1.J3-B8(-J3B-:C/BE1) ; also sheet 1
C/BE2#: X1.J3-D14(-J3D-:C/BE2) ; also sheet 1
C/BE3#: X1.J3-B19(-J3B-:C/BE3) ; also sheet 1
CLK0: X1.J3-B26(-J3B-:CLK0) ; also sheet 1
CLK1: X1.J3-D26(-J3D-:CLK1) ; also sheet 1
CLK2: X1.J3-A27(-J3A-:CLK2) ; also sheet 1
CLK3: X1.J3-C27(-J3C-:CLK3) ; also sheet 1
DEVSEL#: X1.J3-D12(-J3D-:DEVSEL) ; also sheet 1,2
FRAME#: X1.J3-A13(-J3A-:FRAME) ; also sheet 1,2
GND: X1.J3-A1(-J3A-:5.0V/KEY) X1.J3-A5(-J3A-:GND) X1.J3-A10(-J3A-:GND) X1.J3-A14(-J3A-:GND) X1.J3-A20(-J3A-:GND) X1.J3-A24(-J3A-:GND) X1.J3-A28(-J3A-:GND) X1.J3-B3(-J3B-:GND) X1.J3-B9(-J3B-:GND) X1.J3-B13(-J3B-:GND) X1.J3-B18(-J3B-:GND) X1.J3-B23(-J3B-:GND) X1.J3-C4(-J3C-:GND) X1.J3-C7(-J3C-:GND) X1.J3-C12(-J3C-:GND) X1.J3-C16(-J3C-:GND) X1.J3-C22(-J3C-:GND) X1.J3-C26(-J3C-:GND) X1.J3-D5(-J3D-:GND) X1.J3-D6(-J3D-:M66EN) X1.J3-D11(-J3D-:GND) X1.J3-D15(-J3D-:GND) X1.J3-D20(-J3D-:GND) X1.J3-D25(-J3D-:GND) X1.J3-D27(-J3D-:GND) X1.J3-D30(-J3D-:3.3/KEY) ; also sheet 1,2,3,4,5,6,7,12
GNT0#: X1.J3-D24(-J3D-:GNT0) ; also sheet 1
GNT1#: X1.J3-A25(-J3A-:GNT1) ; also sheet 1
GNT2#: X1.J3-C25(-J3C-:GNT2) ; also sheet 1
GNT3#: X1.J3-C30(-J3C-:RESERVED) ; also sheet 1
IDSEL0: X1.J3-A18(-J3A-:IDSEL0) ; also sheet 1
IDSEL1: X1.J3-C18(-J3C-:IDSEL1) ; also sheet 1
IDSEL2: X1.J3-D18(-J3D-:IDSEL2) ; also sheet 1
IDSEL3: X1.J3-D19(-J3D-:IDSEL3) ; also sheet 1
INTA#: X1.J3-B29(-J3B-:INTA) ; also sheet 1,2
INTB#: X1.J3-C29(-J3C-:INTB) ; also sheet 1,2
INTC#: X1.J3-D29(-J3D-:INTC) ; also sheet 1,2
INTD#: X1.J3-B28(-J3B-:INTD) ; also sheet 1,2
IRDY#: X1.J3-C13(-J3C-:IRDY) ; also sheet 1,2
LOCK#: X1.J3-C11(-J3C-:LOCK) ; also sheet 2
PAR: X1.J3-D9(-J3D-:PAR) ; also sheet 1
PERR#: X1.J3-B10(-J3B-:PERR) ; also sheet 1,2
PME#: X1.J3-D10(-J3D-:SDONE) ; also sheet 1
PSON#: X1.J3-C9(-J3C-:SB0) ; also sheet 12
REQ0#: X1.J3-A23(-J3A-:REQ0) ; also sheet 1
REQ1#: X1.J3-C23(-J3C-:REQ1) ; also sheet 1
REQ2#: X1.J3-B24(-J3B-:REQ2) ; also sheet 1
REQ3#: X1.J3-B30(-J3B-:RESERVED) ; also sheet 1
RST#: X1.J3-D28(-J3D-:RST) ; also sheet 1
SERR#: X1.J3-A9(-J3A-:SERR) ; also sheet 1,2
STOP#: X1.J3-A11(-J3A-:STOP) ; also sheet 1,2
TRDY#: X1.J3-B12(-J3B-:TRDY) ; also sheet 1,2
V3V: X1.J3-A8(-J3A-:+3.3V) X1.J3-A12(-J3A-:+3.3V) X1.J3-A17(-J3A-:+3.3V) X1.J3-B11(-J3B-:+3.3V) X1.J3-B15(-J3B-:+3.3V) X1.J3-C10(-J3C-:+3.3V) X1.J3-C14(-J3C-:+3.3V) X1.J3-D8(-J3D-:+3.3V) X1.J3-D13(-J3D-:+3.3V) X1.J3-D17(-J3D-:+3.3V) ; also sheet 12
V5V: X1.J3-A22(-J3A-:+5V) X1.J3-A26(-J3A-:+5V) X1.J3-B21(-J3B-:+5V) X1.J3-B27(-J3B-:+5V) X1.J3-C1(-J3C-:+5V) X1.J3-C24(-J3C-:+5V) X1.J3-C28(-J3C-:+5V) X1.J3-D2(-J3D-:+5V) ; also sheet 12
V5VSB: X1.J3-B1(-J3B-:RESERVED) ; also sheet 12
V12M: X1.J3-A30(-J3A-:-12V) ; also sheet 12
V12P: X1.J3-A29(-J3A-:+12V) ; also sheet 12
VIO: X1.J3-A2(-J3A-:VI/O) X1.J3-B6(-J3B-:VI/O) X1.J3-B25(-J3B-:VI/O) X1.J3-C19(-J3C-:VI/O) X1.J3-D23(-J3D-:VI/O)

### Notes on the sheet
- M66EN

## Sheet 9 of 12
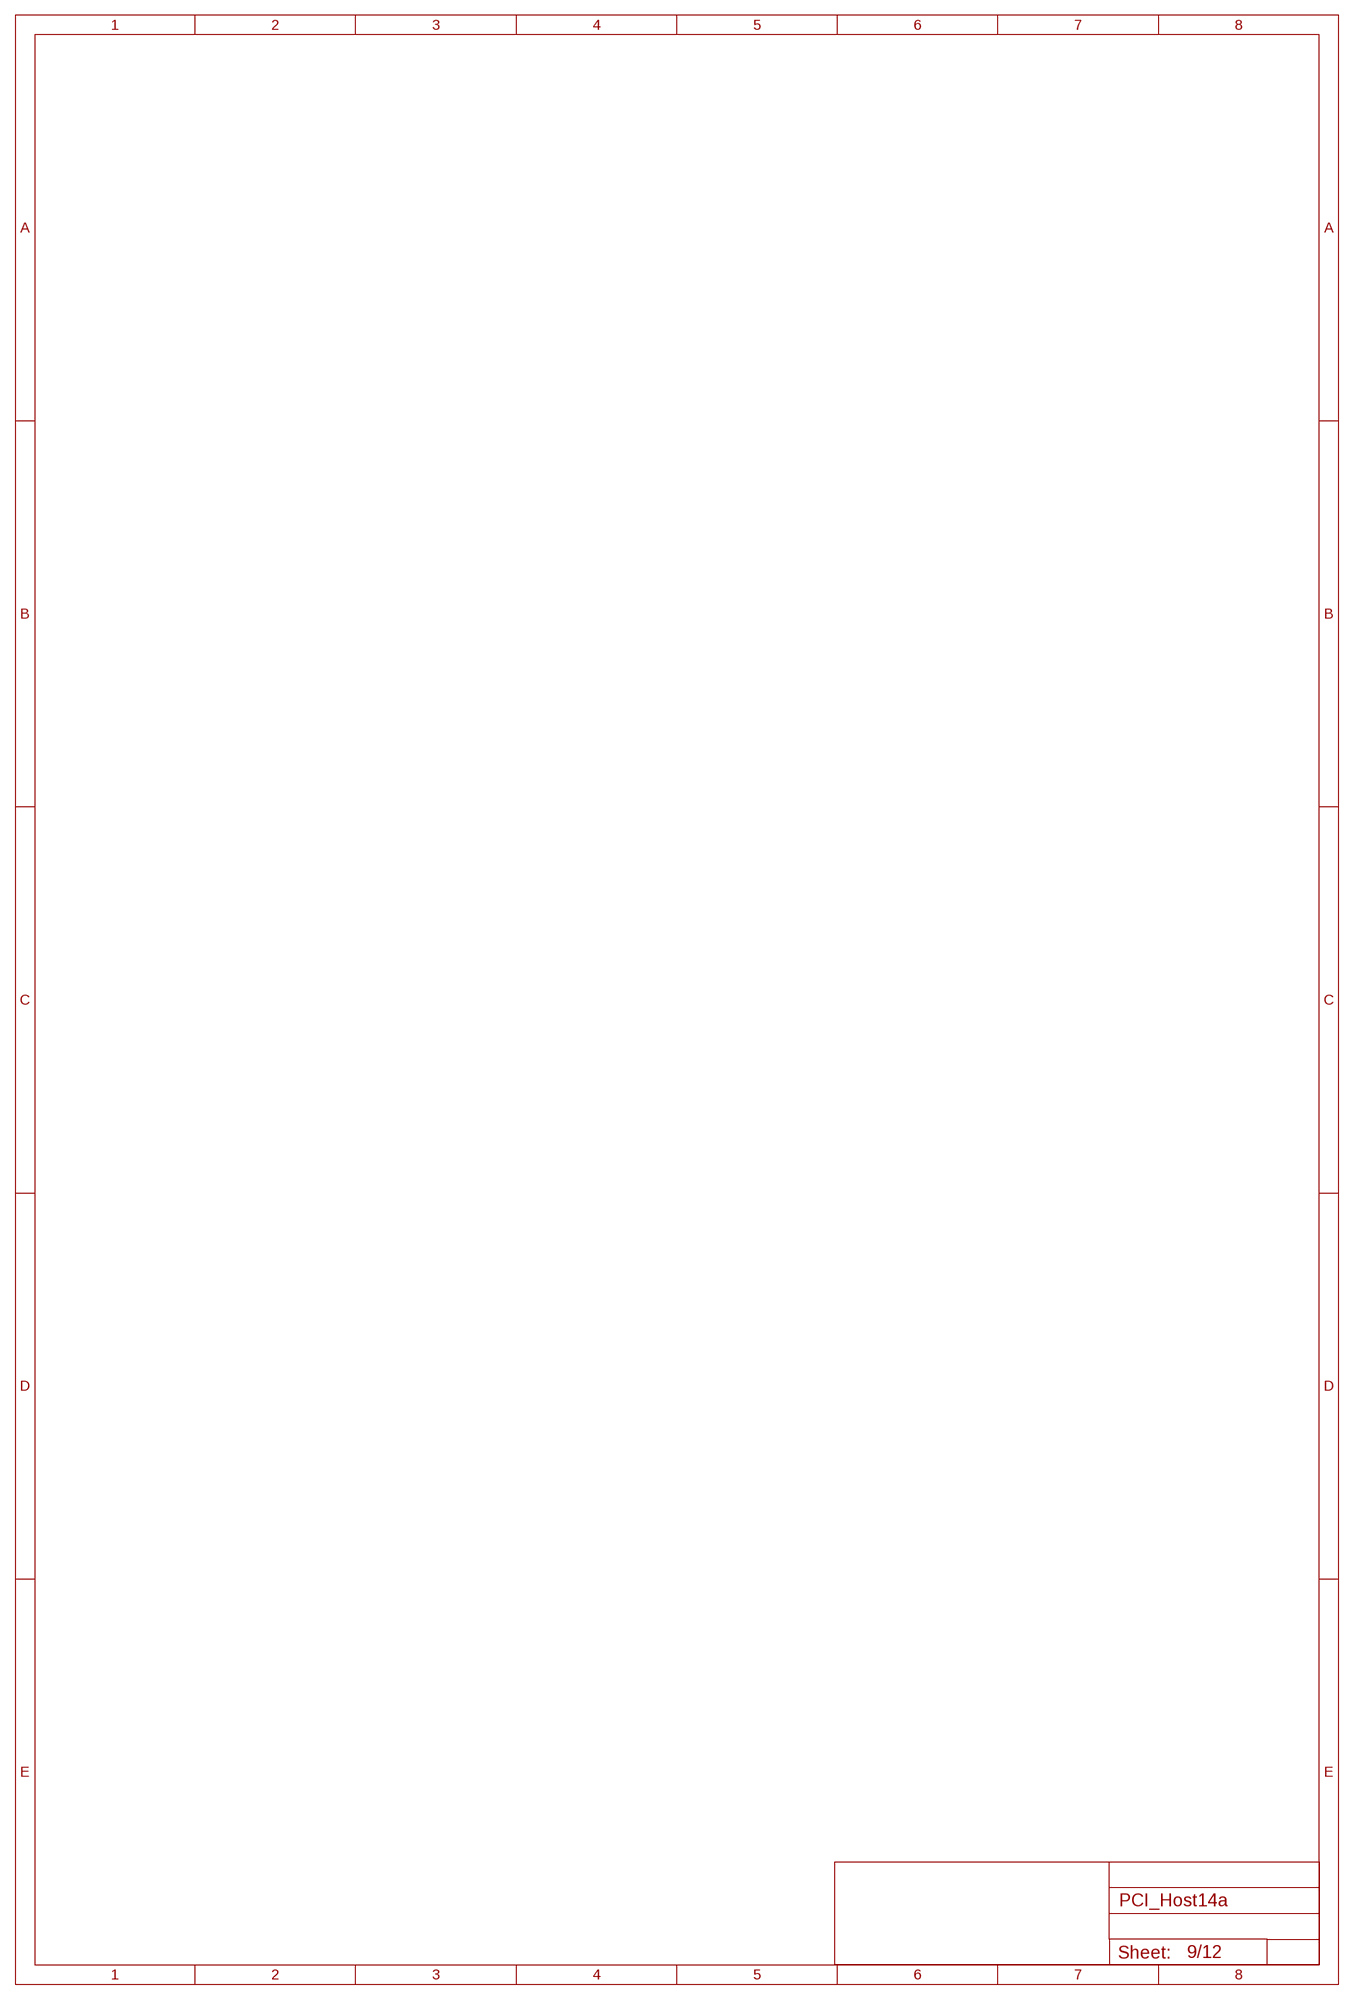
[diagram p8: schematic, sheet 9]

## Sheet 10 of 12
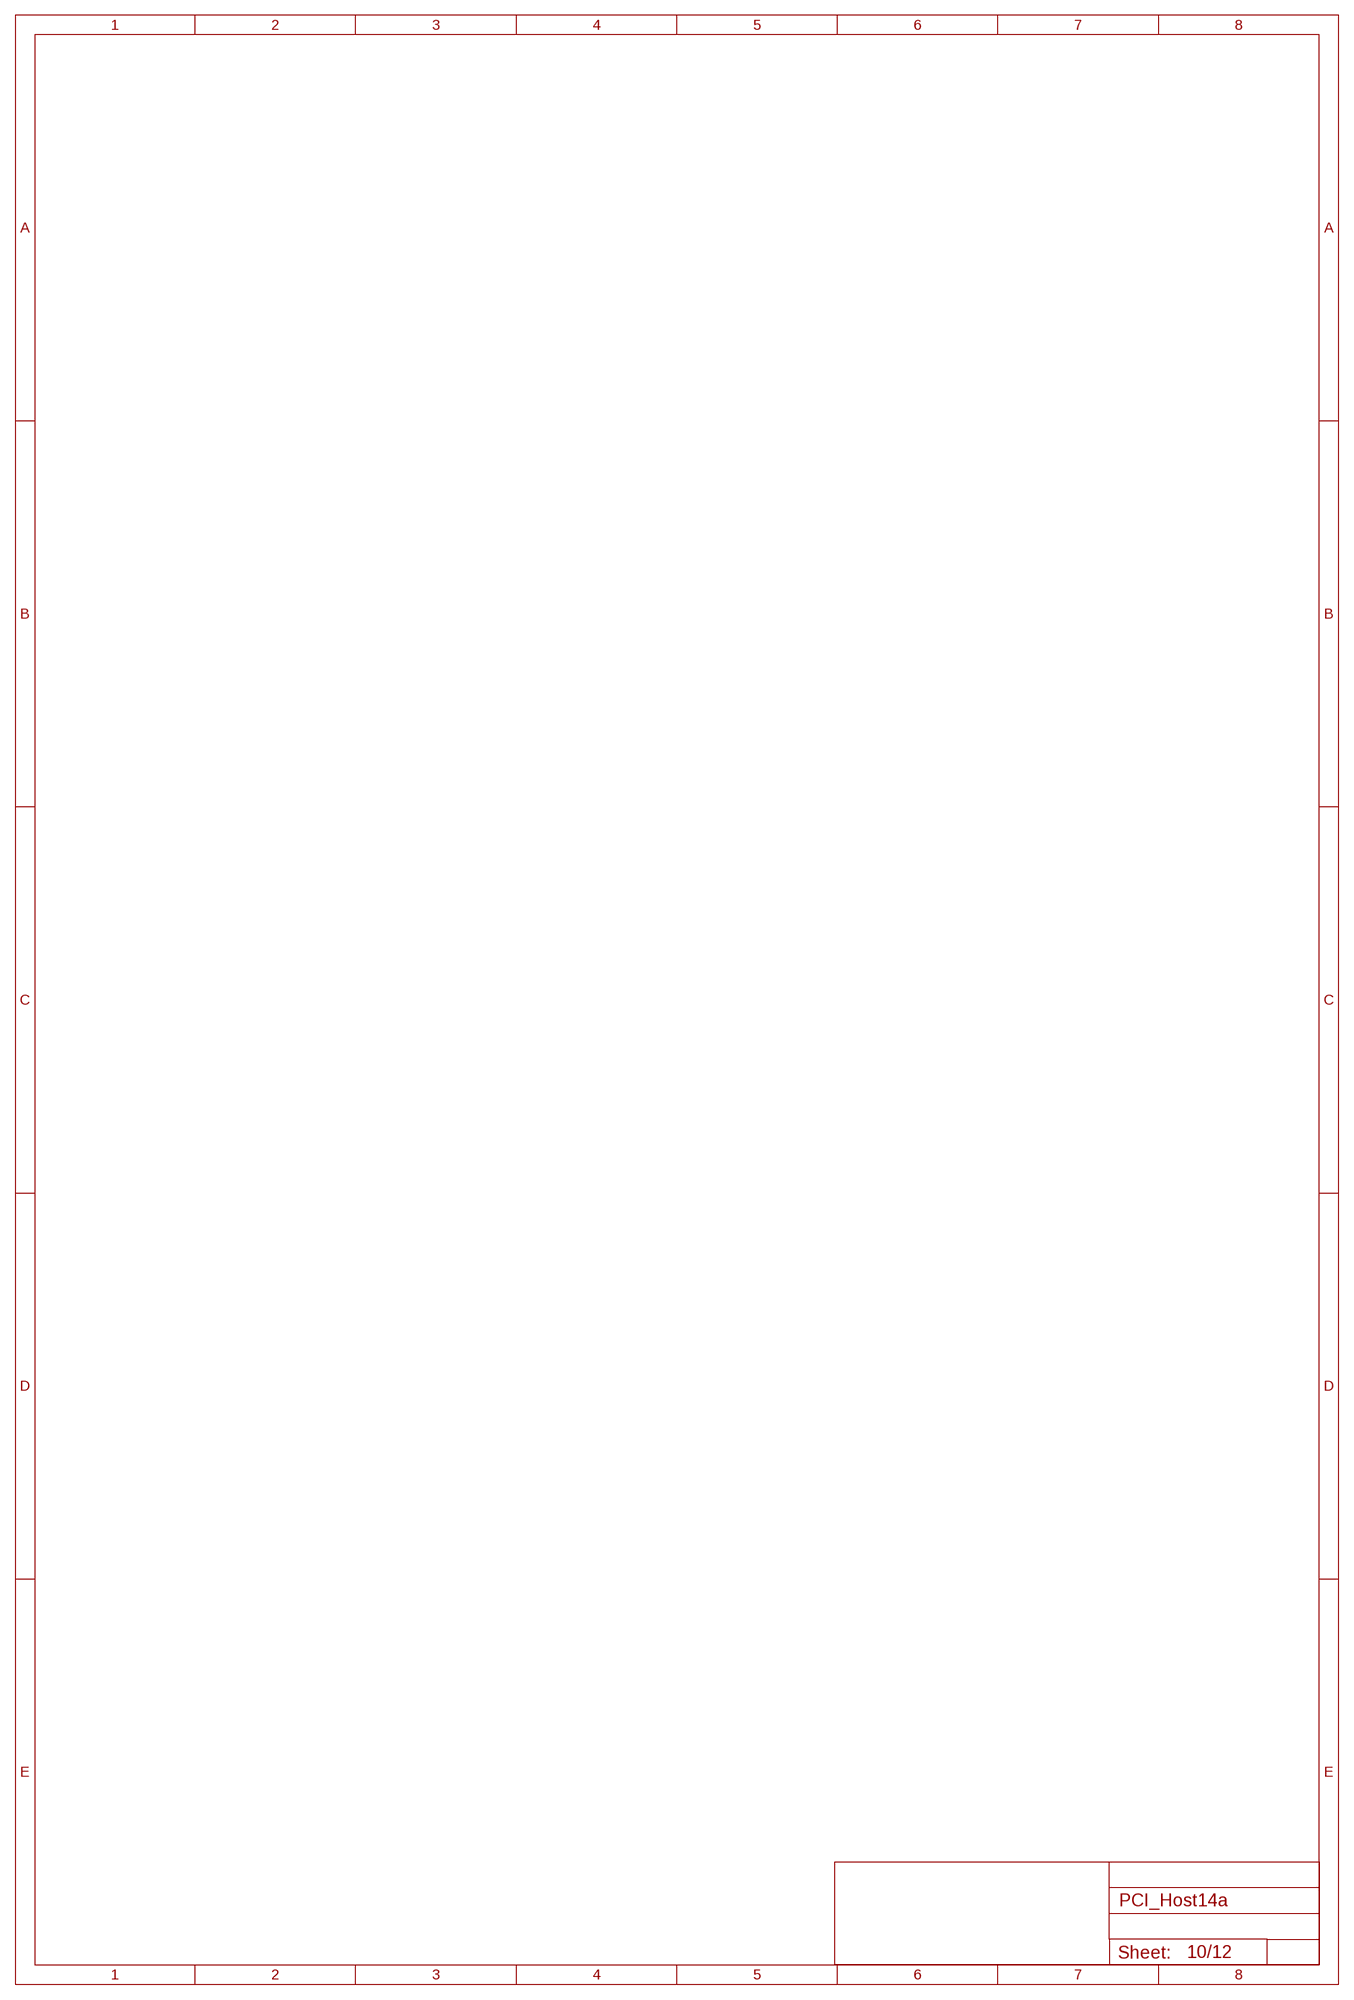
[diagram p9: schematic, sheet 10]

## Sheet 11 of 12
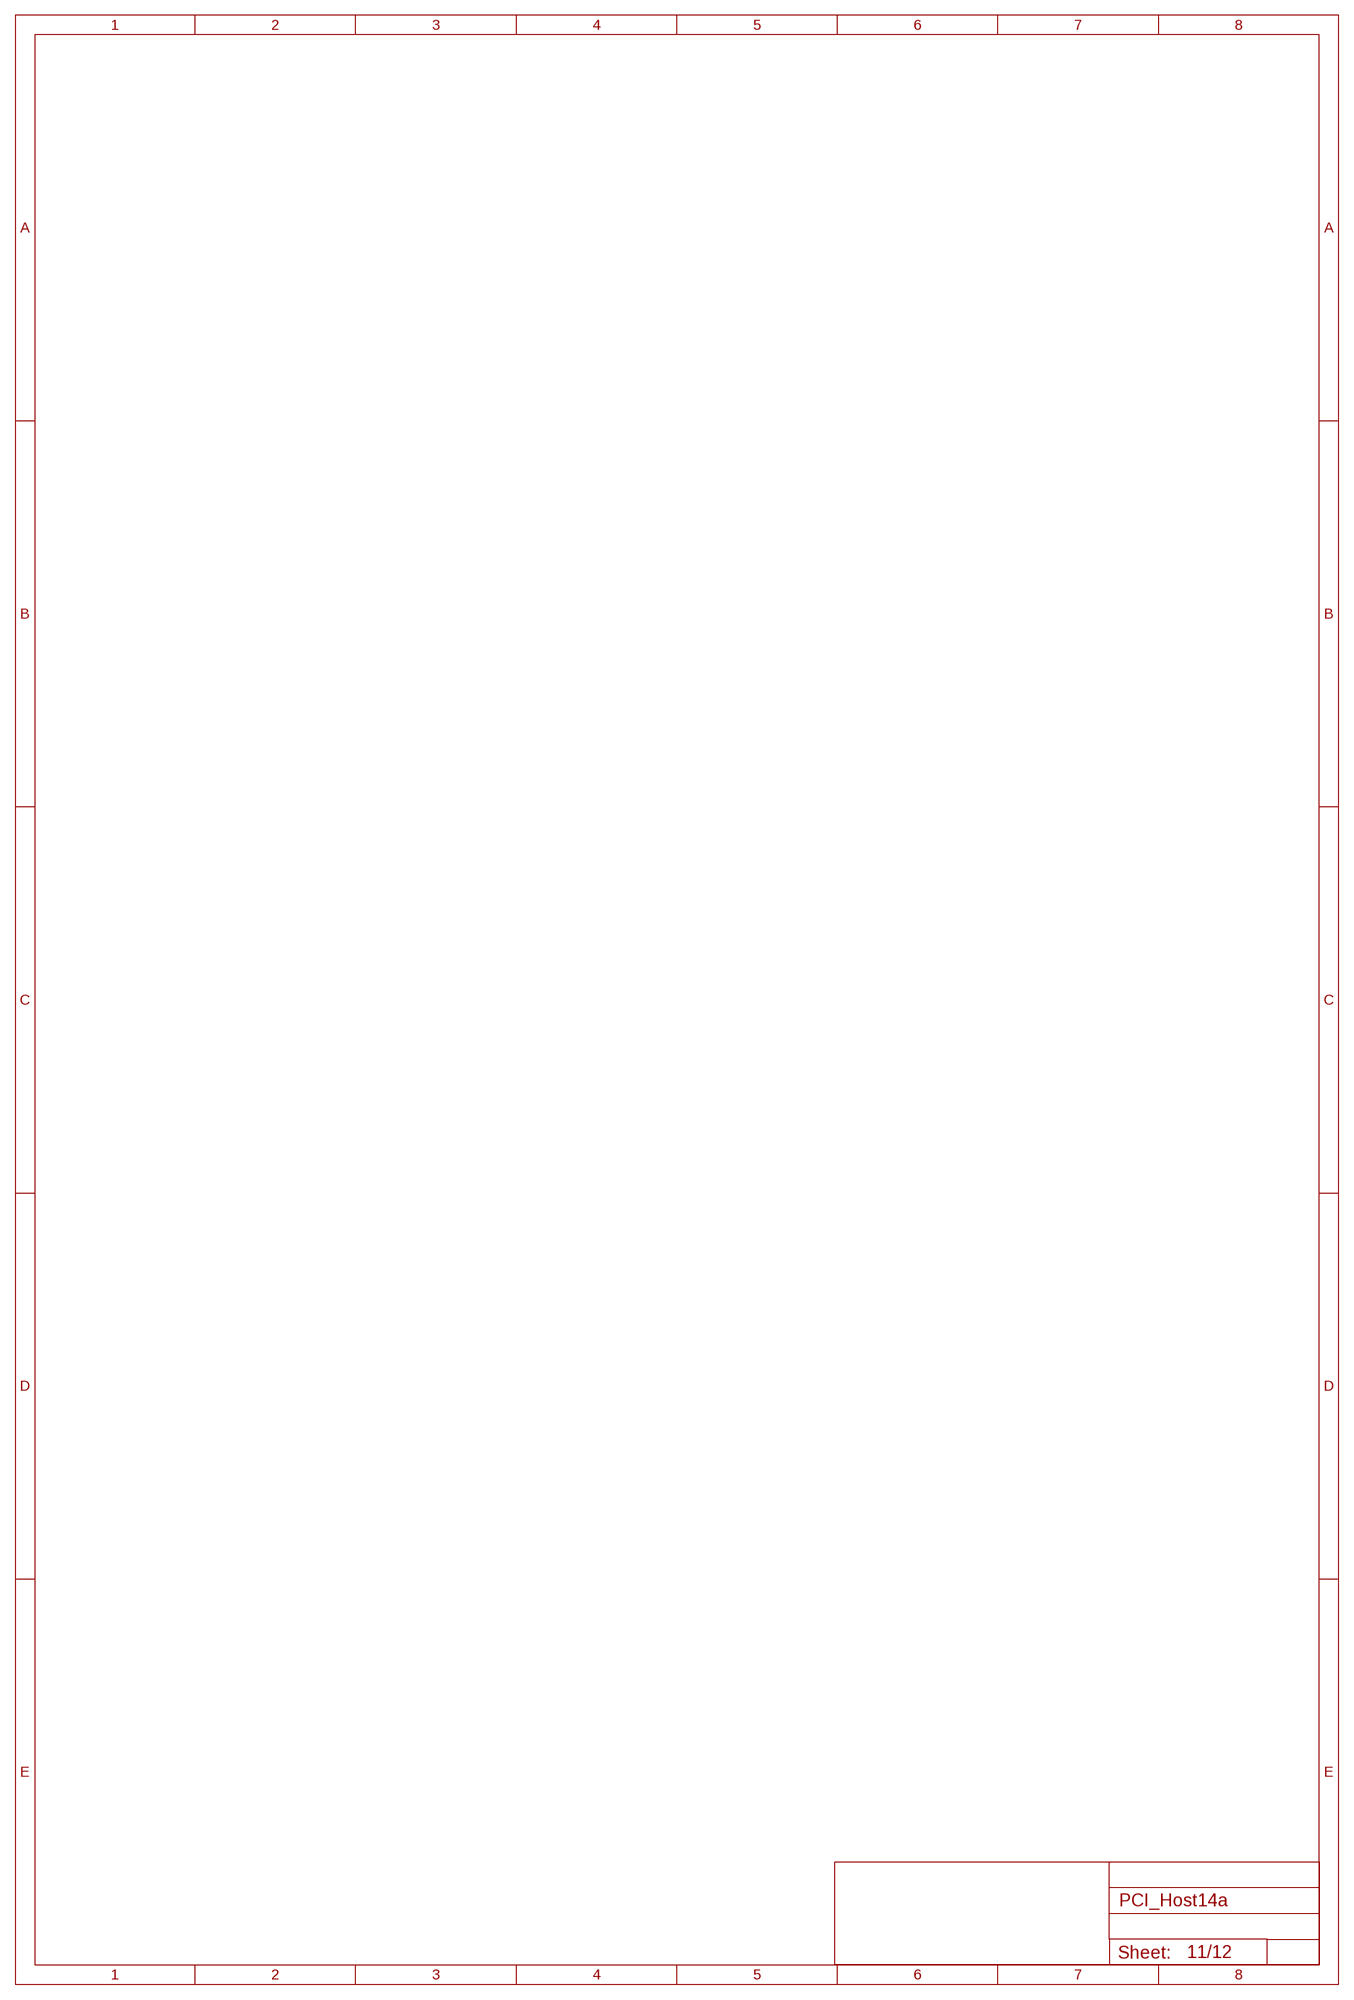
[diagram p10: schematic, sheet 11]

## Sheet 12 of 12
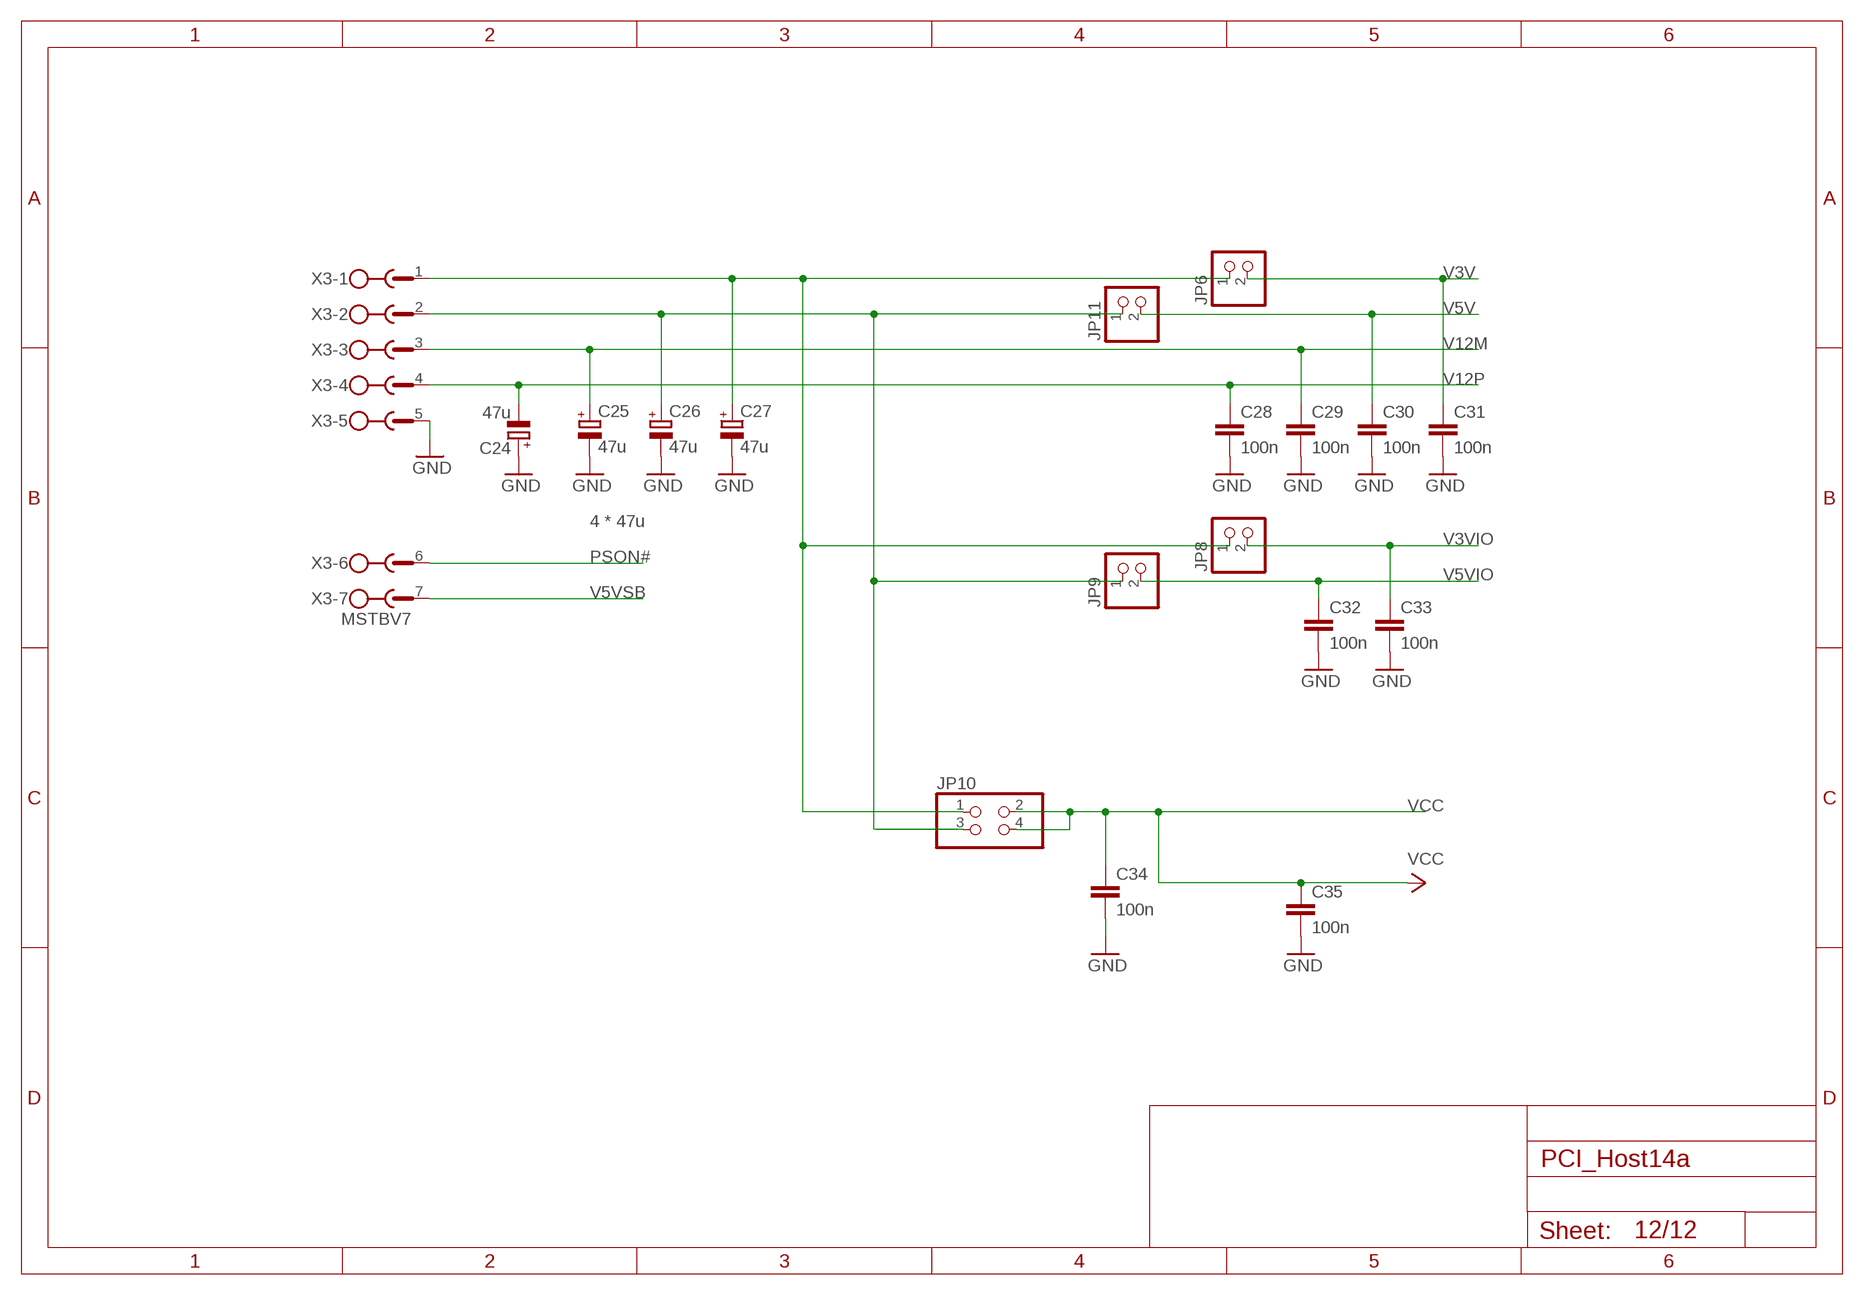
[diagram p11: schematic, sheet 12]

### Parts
C24  47u  CPOL-EUE2.5-6  [E2,5-6]
C25  47u  CPOL-EUE2.5-6  [E2,5-6]
C26  47u  CPOL-EUE2.5-6  [E2,5-6]
C27  47u  CPOL-EUE2.5-6  [E2,5-6]
C28  100n  C-EU025-025X050  [C025-025X050]
C29  100n  C-EU025-025X050  [C025-025X050]
C30  100n  C-EU025-025X050  [C025-025X050]
C31  100n  C-EU025-025X050  [C025-025X050]
C32  100n  C-EU025-025X050  [C025-025X050]
C33  100n  C-EU025-025X050  [C025-025X050]
C34  100n  C-EU025-025X050  [C025-025X050]
C35  100n  C-EU025-025X050  [C025-025X050]
JP6  PINHD-1X2  [1X02]
JP8  PINHD-1X2  [1X02]
JP9  PINHD-1X2  [1X02]
JP10  PINHD-2X2  [2X02]
JP11  PINHD-1X2  [1X02]
X3  MSTBV7  [MSTBV7]

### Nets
GND: C24.+ C25.- C26.- C27.- C28.2 C29.2 C30.2 C31.2 C32.2 C33.2 C34.2 C35.2 X3.5 ; also sheet 1,2,3,4,5,6,7,8
N$10: C26.+ JP9.1 JP10.3 JP11.1 X3.2
N$36: C27.+ JP6.1 JP8.1 JP10.1 X3.1
PSON#: X3.6 ; also sheet 8
V3V: C31.1 JP6.2 ; also sheet 8
V3VIO: C33.1 JP8.2
V5V: C30.1 JP11.2 ; also sheet 8
V5VIO: C32.1 JP9.2
V5VSB: X3.7 ; also sheet 8
V12M: C25.+ C29.1 X3.3 ; also sheet 8
V12P: C24.- C28.1 X3.4 ; also sheet 8
VCC: C34.1 C35.1 JP10.2 JP10.4 ; also sheet 1,2,3,4,5,6,7

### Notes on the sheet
- 4 * 47u

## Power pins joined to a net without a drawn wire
GND: IC2.15(GND)
VCC: IC2.16(VCC)

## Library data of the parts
C1-C17 C19 C28-C35 = rcl:C-EU: CAPACITOR, European symbol
C18 C24-C27 = rcl:CPOL-EU: POLARIZED CAPACITOR, European symbol
IC1 = atmel-2005:ATMEGA*: MICROCONTROLLER 64/128/256 Kbytes FLASH 4 Kbytes EEPROM 8 Kbytes SRAM 86 General Purpose I/O pins 12-channels16-bit PWM 4 x Serial USARTs 16-channels 10-bit A/D
IC2 = maxim:MAX232: RS232 TRANSEIVER; MF: MAXIM; MPN: MAX232ACPE+; OC_FARNELL: 9723773; OC_NEWARK: 68K4544
IC3 = ftdichip:FT232R: Source: http://www.ftdichip.com/Documents/DataSheets/DS_FT232R_v104.pdf; MPN: FT232RL; OC_FARNELL: 1146032; OC_NEWARK: 91K9918
J1-J3 = con-ml:ML6: HARTING; OC_FARNELL: unknown; OC_NEWARK: unknown
J4 J5 = pinhead:PINHD-1X4: PIN HEADER
J6 J7 = con-subd:F09HP: SUB-D; OC_FARNELL: unknown; OC_NEWARK: unknown
J8 = con-ml:ML10: HARTING; OC_FARNELL: unknown; OC_NEWARK: unknown
JP1 JP3 JP5 JP6 JP8 JP9 JP11 = pinhead:PINHD-1X2: PIN HEADER
JP2 = pinhead:PINHD-2X8: PIN HEADER
JP4 JP10 = pinhead:PINHD-2X2: PIN HEADER
JP7 = pinhead:PINHD-2X4: PIN HEADER
JP12 JP13 = pinhead:PINHD-1X3: PIN HEADER
L1 = rcl:L-EU: INDUCTOR, European symbol
LED1-LED4 = led:LED: LED
QG1 = crystal:SM77H: 3.3V CMOS Clock Oscillator Source: www.pletronics.com .. sm77h%203.3v.pdf; OC_FARNELL: unknown; OC_NEWARK: unknown
R1 R2 = resistor-sil:G08R: SIL RESISTOR; OC_FARNELL: unknown; OC_NEWARK: unknown
R3-R9 = rcl:R-EU_: RESISTOR, European symbol
S1 = switch-omron:10-XX: OMRON SWITCH; MPN: B3F-1000; OC_FARNELL: 176432; OC_NEWARK: 36M3542
X1 = con-pc104-usb-subd:PC104_PLUS_USB_SUBD: PC/104-Plus 16 bit
X2 = con-usb:USB: USB Connectors
X3 = con-phoenix-508:MSTBV7: PHOENIX; OC_FARNELL: unknown; OC_NEWARK: unknown

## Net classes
0 default: width 0.152 mm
